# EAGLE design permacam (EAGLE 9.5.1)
AUTHOR: NEAL JACKSON; REV: A; TITLE: PERMAMOTE

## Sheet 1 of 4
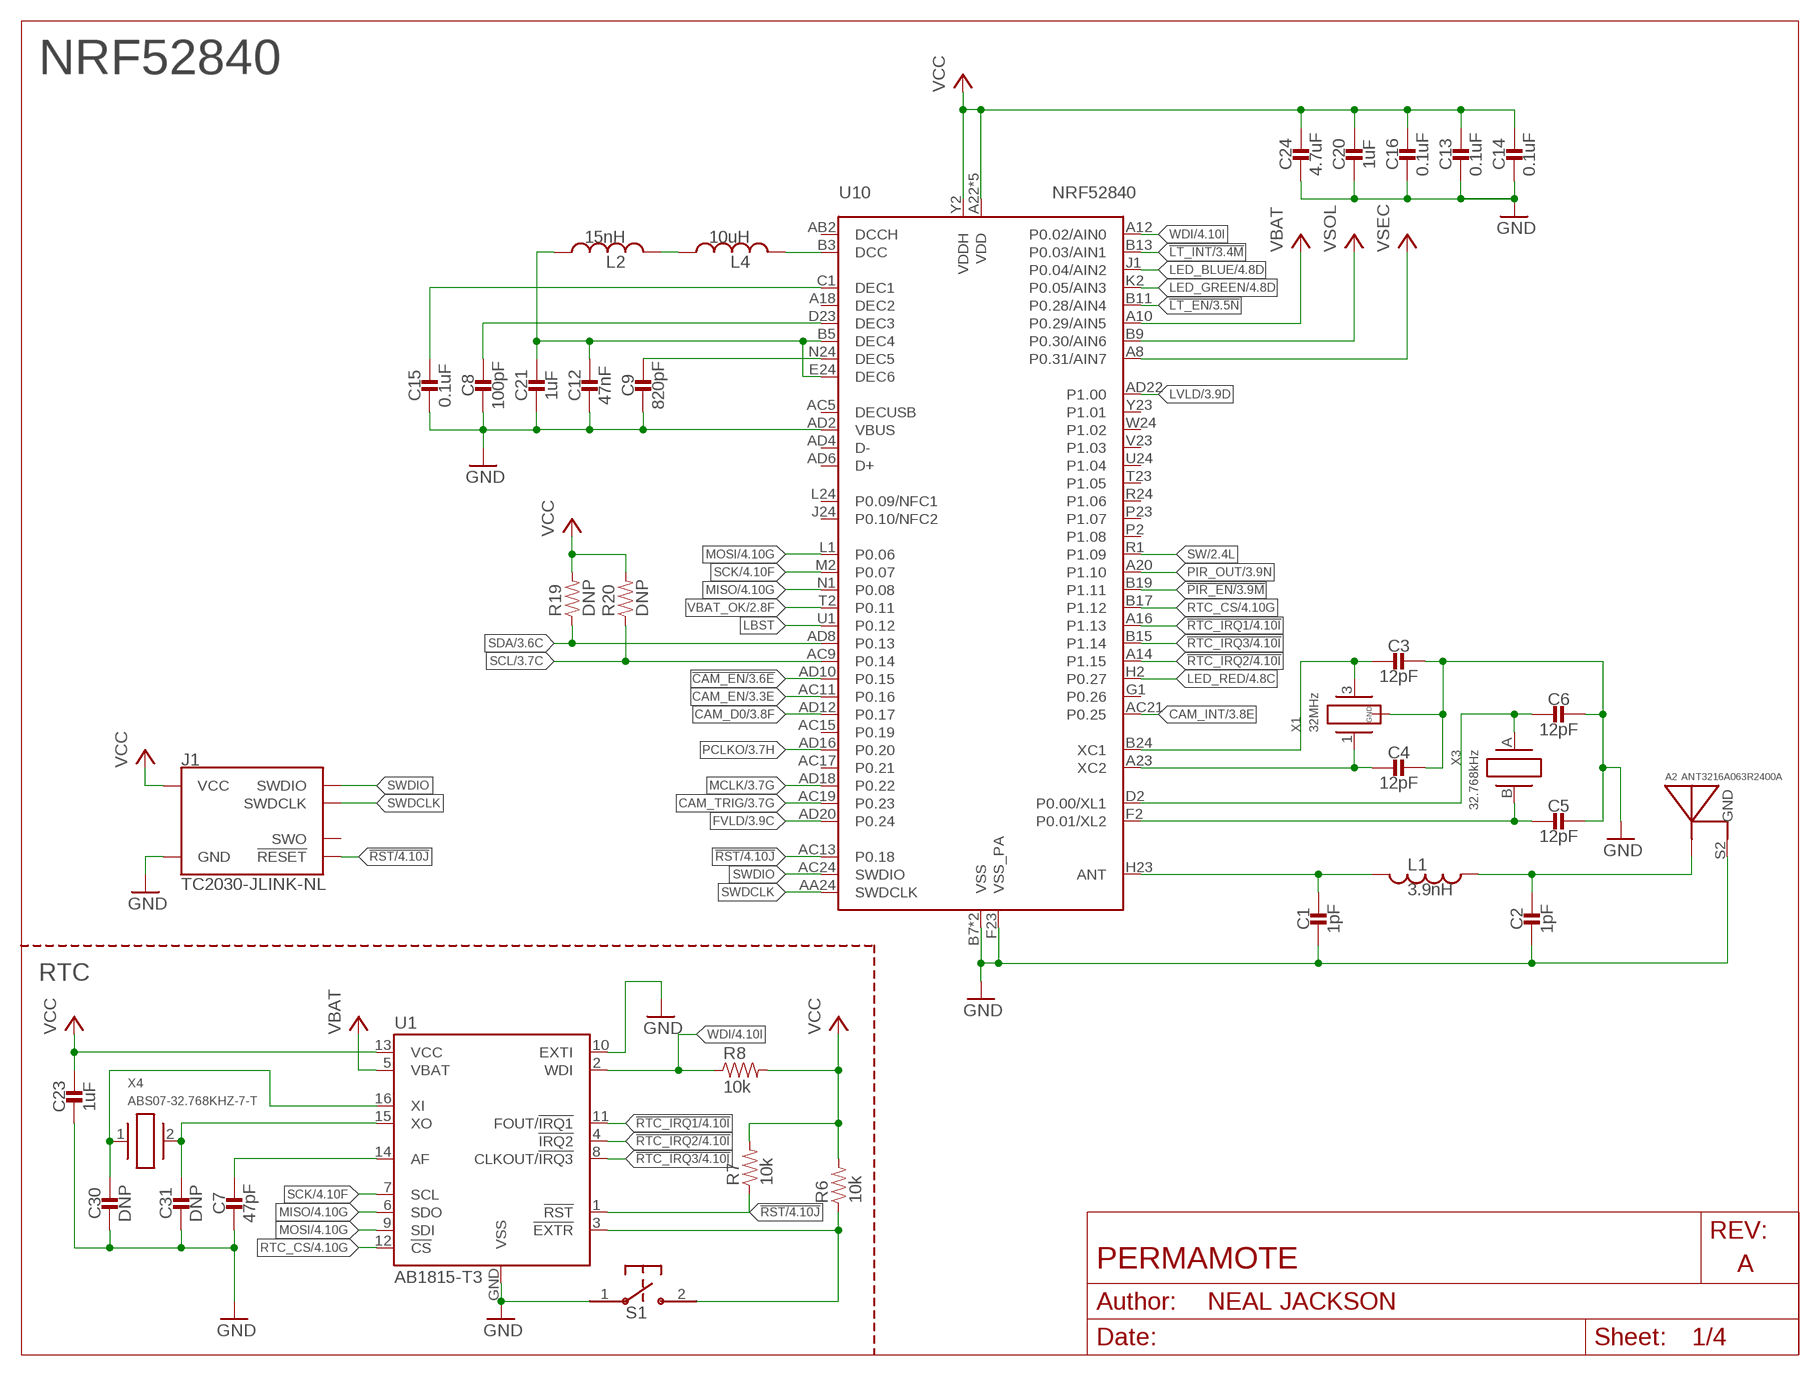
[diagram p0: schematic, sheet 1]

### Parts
A2  ANT3216A063R2400A  [ANT3216A063R2400A]
C1  1pF  CAPACITOR0402_CAP  [0402_CAP]
C2  1pF  CAPACITOR0402_CAP  [0402_CAP]
C3  12pF  CAPACITOR0402_CAP  [0402_CAP]
C4  12pF  CAPACITOR0402_CAP  [0402_CAP]
C5  12pF  CAPACITOR0402_CAP  [0402_CAP]
C6  12pF  CAPACITOR0402_CAP  [0402_CAP]
C7  47pF  CAPACITOR0402_CAP  [0402_CAP]
C8  100pF  CAPACITOR0402_CAP  [0402_CAP]
C9  820pF  CAPACITOR0402_CAP  [0402_CAP]
C12  47nF  CAPACITOR0402_CAP  [0402_CAP]
C13  0.1uF  CAPACITOR0402_CAP  [0402_CAP]
C14  0.1uF  CAPACITOR0402_CAP  [0402_CAP]
C15  0.1uF  CAPACITOR0402_CAP  [0402_CAP]
C16  0.1uF  CAPACITOR0402_CAP  [0402_CAP]
C20  1uF  CAPACITOR0402_CAP  [0402_CAP]
C21  1uF  CAPACITOR0402_CAP  [0402_CAP]
C23  1uF  CAPACITOR0402_CAP  [0402_CAP]
C24  4.7uF  CAPACITOR0402_CAP  [0402_CAP]
C30  DNP  CAPACITOR0402_CAP  [0402_CAP]
C31  DNP  CAPACITOR0402_CAP  [0402_CAP]
J1  TC2030-JLINK-NL  [TC2030-IDC-NL]
L1  3.9nH  INDUCTOR0402  [0402_CAP]
L2  15nH  INDUCTOR0402  [0402_CAP]
L4  10uH  INDUCTOR0603  [0603_CAP]
R6  10k  RESISTOR0402_RES  [0402_RES]
R7  10k  RESISTOR0402_RES  [0402_RES]
R8  10k  RESISTOR0402_RES  [0402_RES]
R19  DNP  RESISTOR0402_RES  [0402_RES]
R20  DNP  RESISTOR0402_RES  [0402_RES]
S1  B3U-1000P  [B3U-1000P]
U1  AB1815-T3  [QFN-16-3MM]
U10  NRF52840  [AQFN73]
X1  32MHz  7V-32.000MAHV-T  [TXC-7V]
X3  32.768kHz  ABS05-32.768KHZ-9-T  [ABS05]
X4  ABS07-32.768KHZ-7-T  [2-SMD]

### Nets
!CAM_EN: U10.AD10(P0.15) ; also sheet 3
!LT_EN: U10.B11(P0.28/AIN4) ; also sheet 3,4
!LT_INT: U10.B13(P0.03/AIN1) ; also sheet 3,4
!PIR_EN: U10.B19(P1.11) ; also sheet 3,4
!RST: J1.3(!RESET) R7.1 U1.1(!RST) U10.AC13(P0.18) ; also sheet 4
!RTC_EXTR: R6.1 S1.2 U1.3(!EXTR)
!RTC_IRQ1: U1.11(FOUT/!IRQ1) U10.A16(P1.13) ; also sheet 4
!RTC_IRQ2: U1.4(!IRQ2) U10.A14(P1.15) ; also sheet 4
!RTC_IRQ3: U1.8(CLKOUT/!IRQ3) U10.B15(P1.14) ; also sheet 4
CAM_D0: U10.AD12(P0.17) ; also sheet 3,4
CAM_EN: U10.AC11(P0.16) ; also sheet 3
CAM_INT: U10.AC21(P0.25) ; also sheet 3
CAM_TRIG: U10.AC19(P0.23) ; also sheet 3
FVLD: U10.AD20(P0.24) ; also sheet 3,4
GND: A2.S2(GND) C1.2 C2.2 C3.1 C4.1 C5.1 C6.1 C7.2 C8.2 C9.2 C12.2 C13.2 C14.2 C15.2 C16.2 C20.2 C21.2 C23.2 C24.2 C30.2 C31.2 J1.5(GND) S1.1 U1.10(EXTI) U1.GND(VSS) U10.AD2(VBUS) U10.B7(VSS) U10.F23(VSS_PA) U10.GND(VSS) X1.2(GND) X1.4(GND) ; also sheet 2,3,4
LBST: U10.U1(P0.12) ; also sheet 2
LED_BLUE: U10.J1(P0.04/AIN2) ; also sheet 4
LED_GREEN: U10.K2(P0.05/AIN3) ; also sheet 4
LED_RED: U10.H2(P0.27) ; also sheet 4
LVLD: U10.AD22(P1.00) ; also sheet 3,4
MCLK: U10.AD18(P0.22) ; also sheet 3,4
MISO: U1.6(SDO) U10.N1(P0.08) ; also sheet 4
MOSI: U1.9(SDI) U10.L1(P0.06) ; also sheet 4
N$1: C9.1 U10.N24(DEC5)
N$2: C15.1 U10.C1(DEC1)
N$3: C12.1 C21.1 L2.1 U10.B5(DEC4) U10.E24(DEC6)
N$4: C8.1 U10.D23(DEC3)
N$5: C1.1 L1.2 U10.H23(ANT)
N$6: A2.S1(ANTENNA) C2.1 L1.1
N$8: C3.2 U10.B24(XC1) X1.3
N$9: C4.2 U10.A23(XC2) X1.1
N$25: C7.1 U1.14(AF)
N$26: C30.1 U1.16(XI) X4.1
N$27: C31.1 U1.15(XO) X4.2
N$44: L4.2 U10.B3(DCC)
N$49: L2.2 L4.1
PCLKO: U10.AD16(P0.20) ; also sheet 3,4
PIR_OUT: U10.A20(P1.10) ; also sheet 3,4
RTC_CS: U1.12(!CS) U10.B17(P1.12) ; also sheet 4
SCK: U1.7(SCL) U10.M2(P0.07) ; also sheet 4
SCL: R20.1 U10.AC9(P0.14) ; also sheet 3,4
SDA: R19.1 U10.AD8(P0.13) ; also sheet 3,4
SW: U10.R1(P1.09) ; also sheet 2,4
SWDCLK: J1.4(SWDCLK) U10.AA24(SWDCLK)
SWDIO: J1.2(SWDIO) U10.AC24(SWDIO)
VBAT: U1.5(VBAT) U10.A10(P0.29/AIN5) ; also sheet 2
VBAT_OK: U10.T2(P0.11) ; also sheet 2
VCC: C13.1 C14.1 C16.1 C20.1 C23.1 C24.1 J1.1(VCC) R6.2 R7.2 R8.2 R19.2 R20.2 U1.13(VCC) U10.A22(VDD) U10.AD14(VDD) U10.AD23(VDD) U10.B1(VDD) U10.W1(VDD) U10.Y2(VDDH) ; also sheet 2,3,4
VSEC: U10.A8(P0.31/AIN7) ; also sheet 2
VSOL: U10.B9(P0.30/AIN6) ; also sheet 2,4
WDI: R8.1 U1.2(WDI) U10.A12(P0.02/AIN0) ; also sheet 4
XL1: C6.2 U10.D2(P0.00/XL1) X3.A
XL2: C5.2 U10.F2(P0.01/XL2) X3.B
Unconnected: J1.6(SWO) U10.A18(DEC2) U10.AB2(DCCH) U10.AC5(DECUSB) U10.AC15(P0.19) U10.AC17(P0.21) U10.AD4(D-) U10.AD6(D+) U10.G1(P0.26) U10.J24(P0.10/NFC2) U10.L24(P0.09/NFC1) U10.P2(P1.08) U10.P23(P1.07) U10.R24(P1.06) U10.T23(P1.05) U10.U24(P1.04) U10.V23(P1.03) U10.W24(P1.02) U10.Y23(P1.01)

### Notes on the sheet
- NRF52840
- RTC

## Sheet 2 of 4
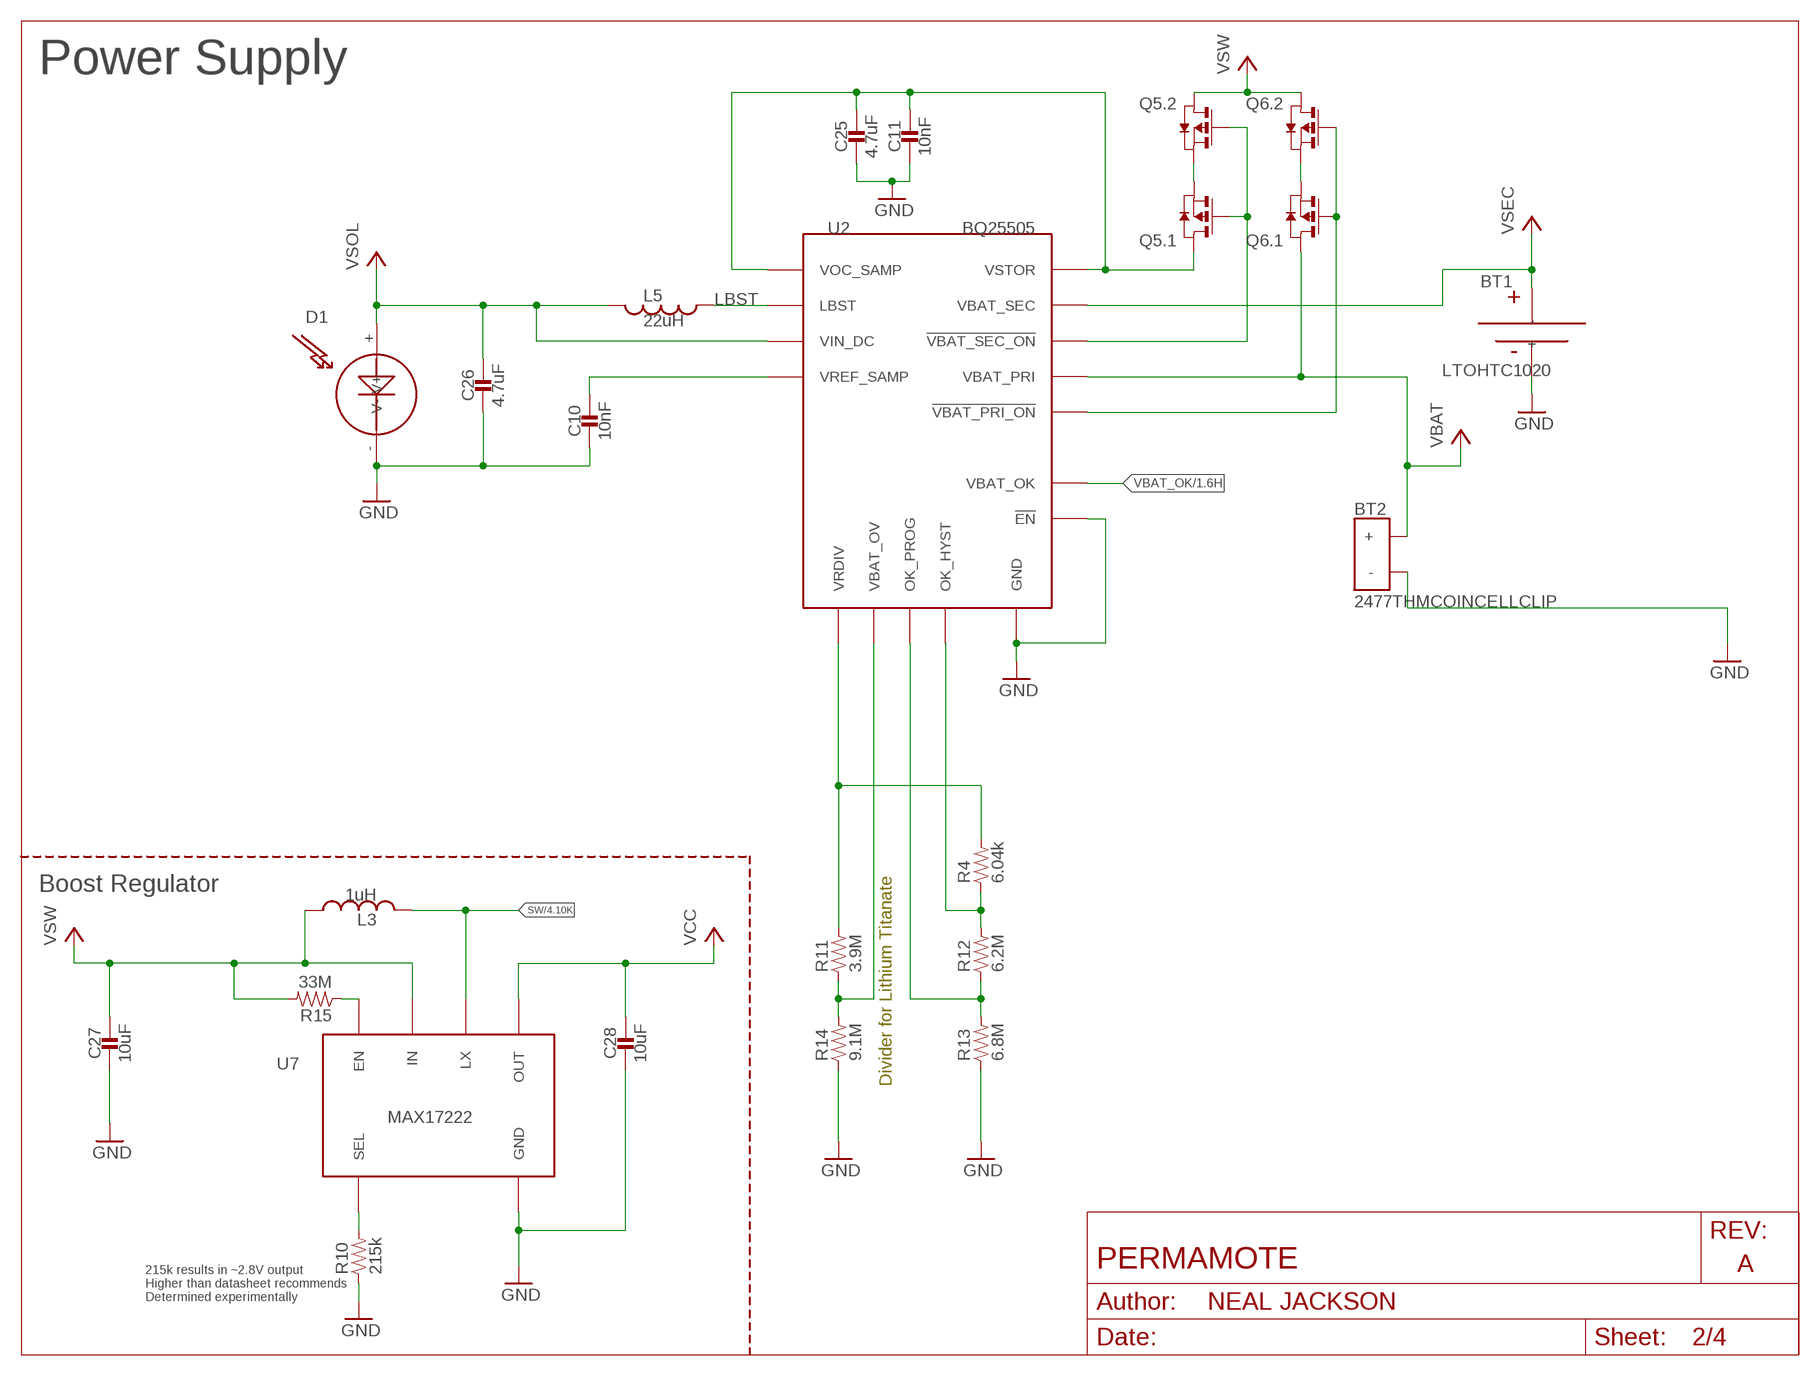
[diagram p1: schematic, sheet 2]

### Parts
BT1  LTOHTC1020  [1020]
BT2  2477THMCOINCELLCLIP  [2477THMCOINCLIP]
C10  10nF  CAPACITOR0402_CAP  [0402_CAP]
C11  10nF  CAPACITOR0402_CAP  [0402_CAP]
C25  4.7uF  CAPACITOR0402_CAP  [0402_CAP]
C26  4.7uF  CAPACITOR0402_CAP  [0402_CAP]
C27  10uF  CAPACITOR0603_CAP  [0603_CAP]
C28  10uF  CAPACITOR0603_CAP  [0603_CAP]
D1  SOLARCELLHOLES  [SOLAR_HOLES]
L3  1uH  INDUCTORIHL  [IHL-1212BZ-11]
L5  22uH  INDUCTOR74437324220  [74437324220]
Q5  PMDXB950UPEL  [XDFN-6]
Q6  PMDXB950UPEL  [XDFN-6]
R4  6.04k  RESISTOR0402_RES  [0402_RES]
R10  215k  RESISTOR0603_RES  [0603-RES]
R11  3.9M  RESISTOR0402_RES  [0402_RES]
R12  6.2M  RESISTOR0402_RES  [0402_RES]
R13  6.8M  RESISTOR0402_RES  [0402_RES]
R14  9.1M  RESISTOR0402_RES  [0402_RES]
R15  33M  RESISTOR0603_RES  [0603-RES]
U2  BQ25505  [S-PVQFN-N20-RGR]
U7  MAX17222  [UDFN-6-MAXIM]

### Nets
!VBAT_PRI_ON: Q6.2(.1:G) Q6.5(.2:G) U2.10(!VBAT_PRI_ON)
!VBAT_SEC_ON: Q5.2(.1:G) Q5.5(.2:G) U2.9(!VBAT_SEC_ON)
GND: BT1.- BT2.GND(-) C10.2 C11.2 C25.2 C26.2 C27.2 C28.2 D1.-(V-) R10.1 R13.1 R14.1 U2.1(GND) U2.5(!EN) U2.6(GND) U2.15(GND) U2.16(GND) U2.17(GND) U2.PAD(GND) U7.3(GND) ; also sheet 1,3,4
LBST: L5.P$1 U2.20(LBST) ; also sheet 1
N$12: R10.2 U7.4(SEL)
N$14: R15.1 U7.6(EN)
N$18: R11.1 R14.2 U2.7(VBAT_OV)
N$32: R4.2 R11.2 U2.8(VRDIV)
N$45: Q5.1(.1:S) Q5.4(.2:S)
N$53: Q6.1(.1:S) Q6.4(.2:S)
N$57: R12.1 R13.2 U2.12(OK_PROG)
N$58: R4.1 R12.2 U2.11(OK_HYST)
SW: L3.P$2 U7.2(LX) ; also sheet 1,4
VBAT: BT2.1(+) BT2.2(+) Q6.6(.1:D) U2.14(VBAT_PRI) ; also sheet 1
VBAT_OK: U2.13(VBAT_OK) ; also sheet 1
VCC: C28.1 U7.1(OUT) ; also sheet 1,3,4
VOC_SAMP_VSTOR: C11.1 C25.1 Q5.6(.1:D) U2.3(VOC_SAMP) U2.19(VSTOR)
VREF_SAMP: C10.1 U2.4(VREF_SAMP)
VSEC: BT1.+ U2.18(VBAT_SEC) ; also sheet 1
VSOL: C26.1 D1.+(V+) L5.P$2 U2.2(VIN_DC) ; also sheet 1,4
VSW: C27.1 L3.P$1 Q5.3(.2:D) Q6.3(.2:D) R15.2 U7.5(IN)

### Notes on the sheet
- Power Supply
- Boost Regulator
- Divider for Lithium Titanate
- 215k results in ~2.8V output
  Higher than datasheet recommends
  Determined experimentally

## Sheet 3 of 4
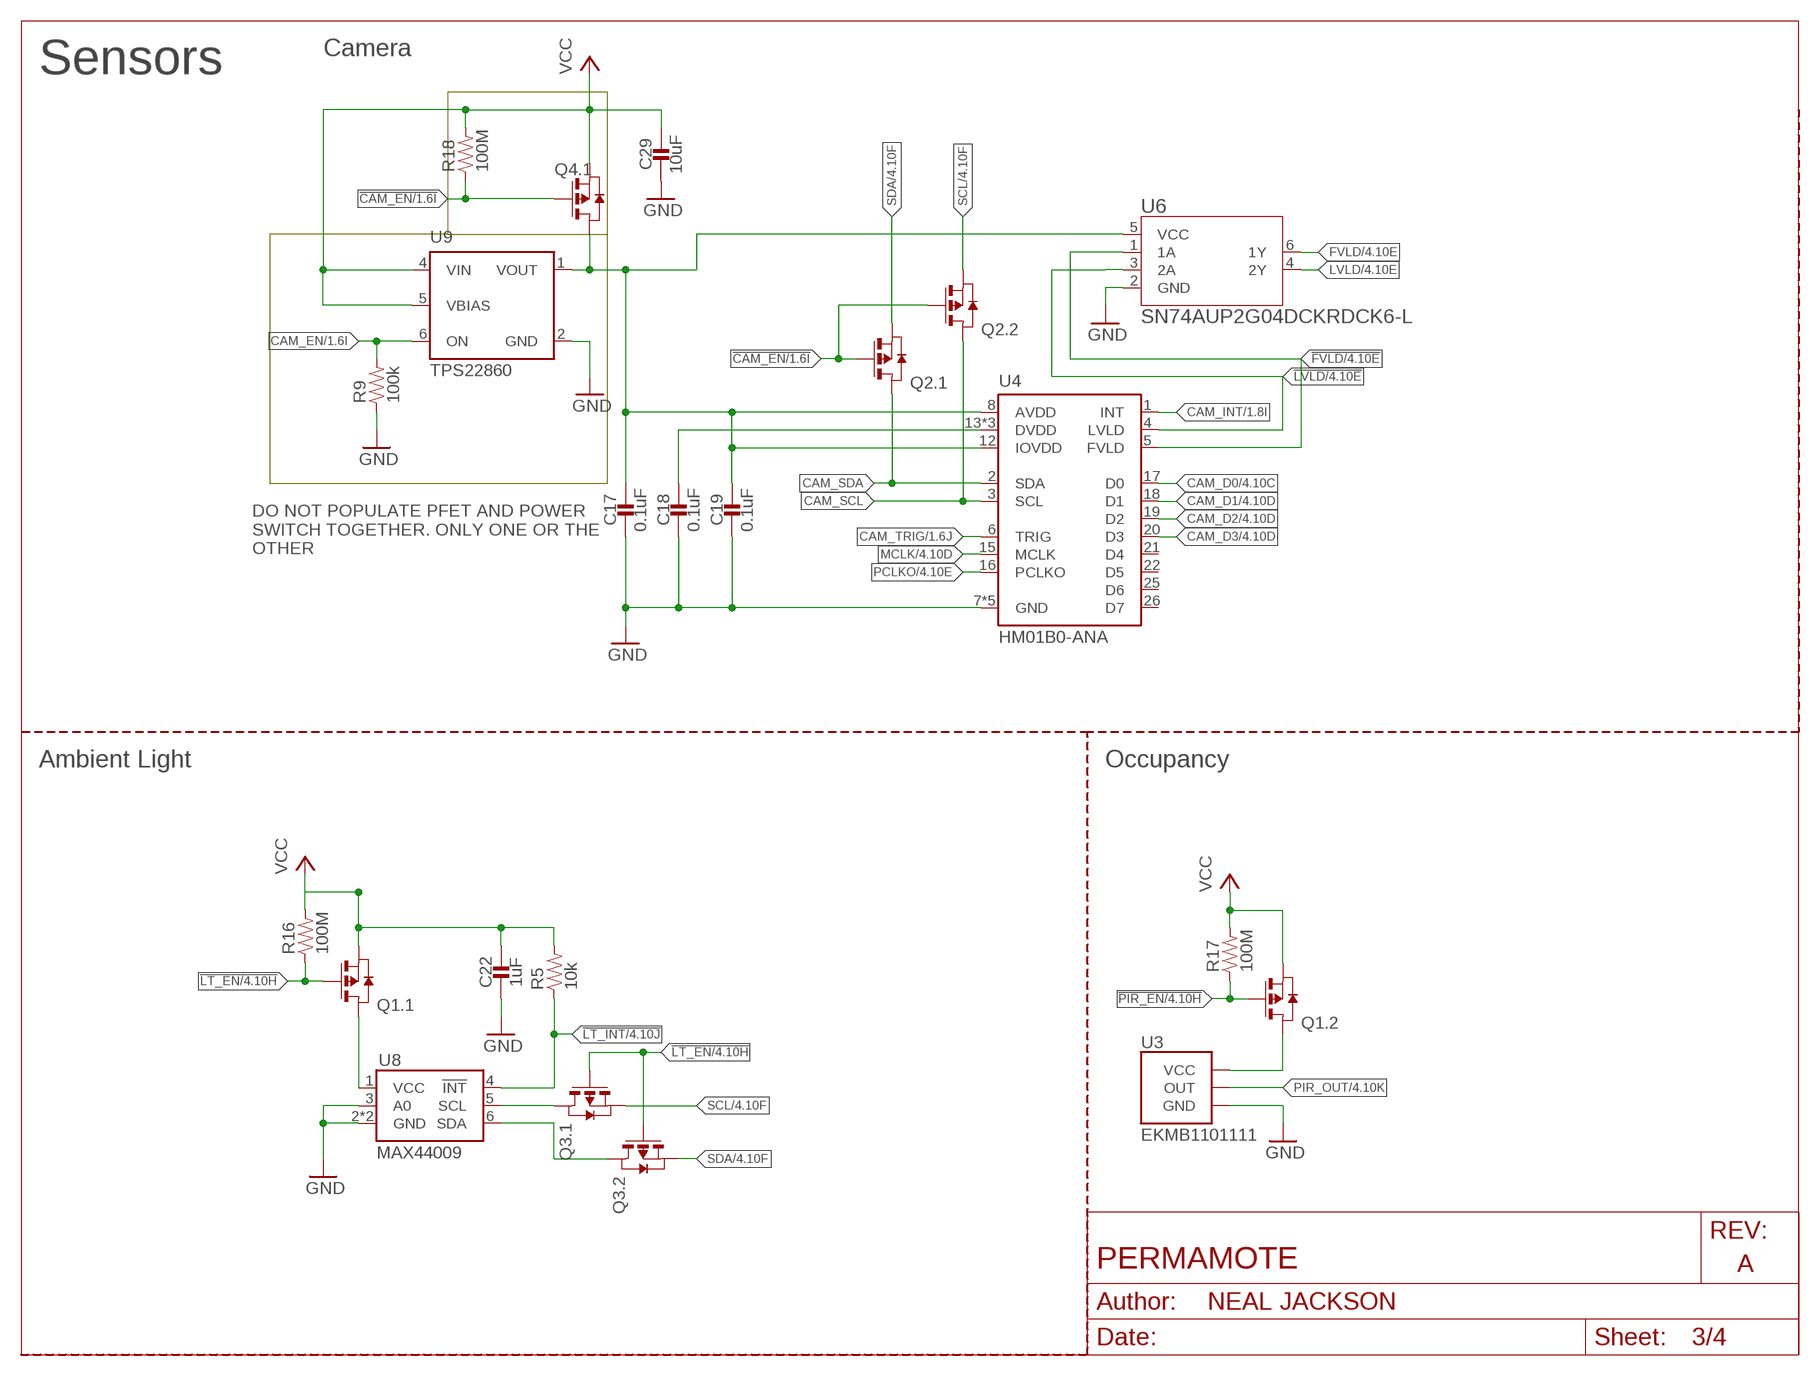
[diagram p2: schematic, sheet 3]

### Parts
C17  0.1uF  CAPACITOR0402_CAP  [0402_CAP]
C18  0.1uF  CAPACITOR0402_CAP  [0402_CAP]
C19  0.1uF  CAPACITOR0402_CAP  [0402_CAP]
C22  1uF  CAPACITOR0402_CAP  [0402_CAP]
C29  10uF  CAPACITOR0603_CAP  [0603_CAP]
Q1  PMDXB950UPEL  [XDFN-6]
Q2  PMDXB950UPEL  [XDFN-6]
Q3  PMDXB950UPEL  [XDFN-6]
Q4  PMDXB950UPEL  [XDFN-6]
R5  10k  RESISTOR0402_RES  [0402_RES]
R9  100k  RESISTOR0402_RES  [0402_RES]
R16  100M  RESISTOR0402_RES  [0402_RES]
R17  100M  RESISTOR0402_RES  [0402_RES]
R18  100M  RESISTOR0402_RES  [0402_RES]
U3  EKMB1101111  [AMN2]
U4  HM01B0-ANA  [NEOPAC-26]
U6  SN74AUP2G04DCKRDCK6-L  [DCK6-L]
U8  MAX44009  [UDFN-6-EXPOSED]
U9  TPS22860  [SOT-23-6]

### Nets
!CAM_EN: Q2.2(.1:G) Q2.5(.2:G) Q4.2(.1:G) R18.1 ; also sheet 1
!FVLD: U4.5(FVLD) U6.1(1A) ; also sheet 4
!LT_EN: Q1.2(.1:G) Q3.2(.1:G) Q3.5(.2:G) R16.1 ; also sheet 1,4
!LT_INT: R5.1 U8.4(!INT) ; also sheet 1,4
!LVLD: U4.4(LVLD) U6.3(2A) ; also sheet 4
!PIR_EN: Q1.5(.2:G) R17.1 ; also sheet 1,4
CAM_D0: U4.17(D0) ; also sheet 1,4
CAM_D1: U4.18(D1) ; also sheet 4
CAM_D2: U4.19(D2) ; also sheet 4
CAM_D3: U4.20(D3) ; also sheet 4
CAM_EN: R9.2 U9.6(ON) ; also sheet 1
CAM_INT: U4.1(INT) ; also sheet 1
CAM_SCL: Q2.3(.2:D) U4.3(SCL)
CAM_SDA: Q2.6(.1:D) U4.2(SDA)
CAM_TRIG: U4.6(TRIG) ; also sheet 1
FVLD: U6.6(1Y) ; also sheet 1,4
GND: C17.2 C18.2 C19.2 C22.2 C29.2 R9.1 U3.GND U4.7(GND) U4.9(GND) U4.10(GND) U4.11(GND) U4.24(GND) U6.2(GND) U8.2(GND) U8.3(A0) U8.EP(GND) U9.2(GND) ; also sheet 1,2,4
LVLD: U6.4(2Y) ; also sheet 1,4
MCLK: U4.15(MCLK) ; also sheet 1,4
N$10: C18.1 U4.13(DVDD) U4.14(DVDD) U4.23(DVDD)
N$13: C17.1 C19.1 Q4.6(.1:D) U4.8(AVDD) U4.12(IOVDD) U6.5(VCC) U9.1(VOUT)
N$20: Q1.6(.1:D) U8.1(VCC)
N$23: Q1.3(.2:D) U3.VCC
N$51: Q3.3(.2:D) U8.6(SDA)
N$52: Q3.6(.1:D) U8.5(SCL)
PCLKO: U4.16(PCLKO) ; also sheet 1,4
PIR_OUT: U3.OUT ; also sheet 1,4
SCL: Q2.4(.2:S) Q3.1(.1:S) ; also sheet 1,4
SDA: Q2.1(.1:S) Q3.4(.2:S) ; also sheet 1,4
VCC: C22.1 C29.1 Q1.1(.1:S) Q1.4(.2:S) Q4.1(.1:S) R5.2 R16.2 R17.2 R18.2 U9.4(VIN) U9.5(VBIAS) ; also sheet 1,2,4
Unconnected: Q4.3(.2:D) Q4.4(.2:S) Q4.5(.2:G) U4.21(D4) U4.22(D5) U4.25(D6) U4.26(D7)

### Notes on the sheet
- Camera
- Sensors
- DO NOT POPULATE PFET AND POWER
  SWITCH TOGETHER. ONLY ONE OR THE
  OTHER
- Ambient Light | Occupancy

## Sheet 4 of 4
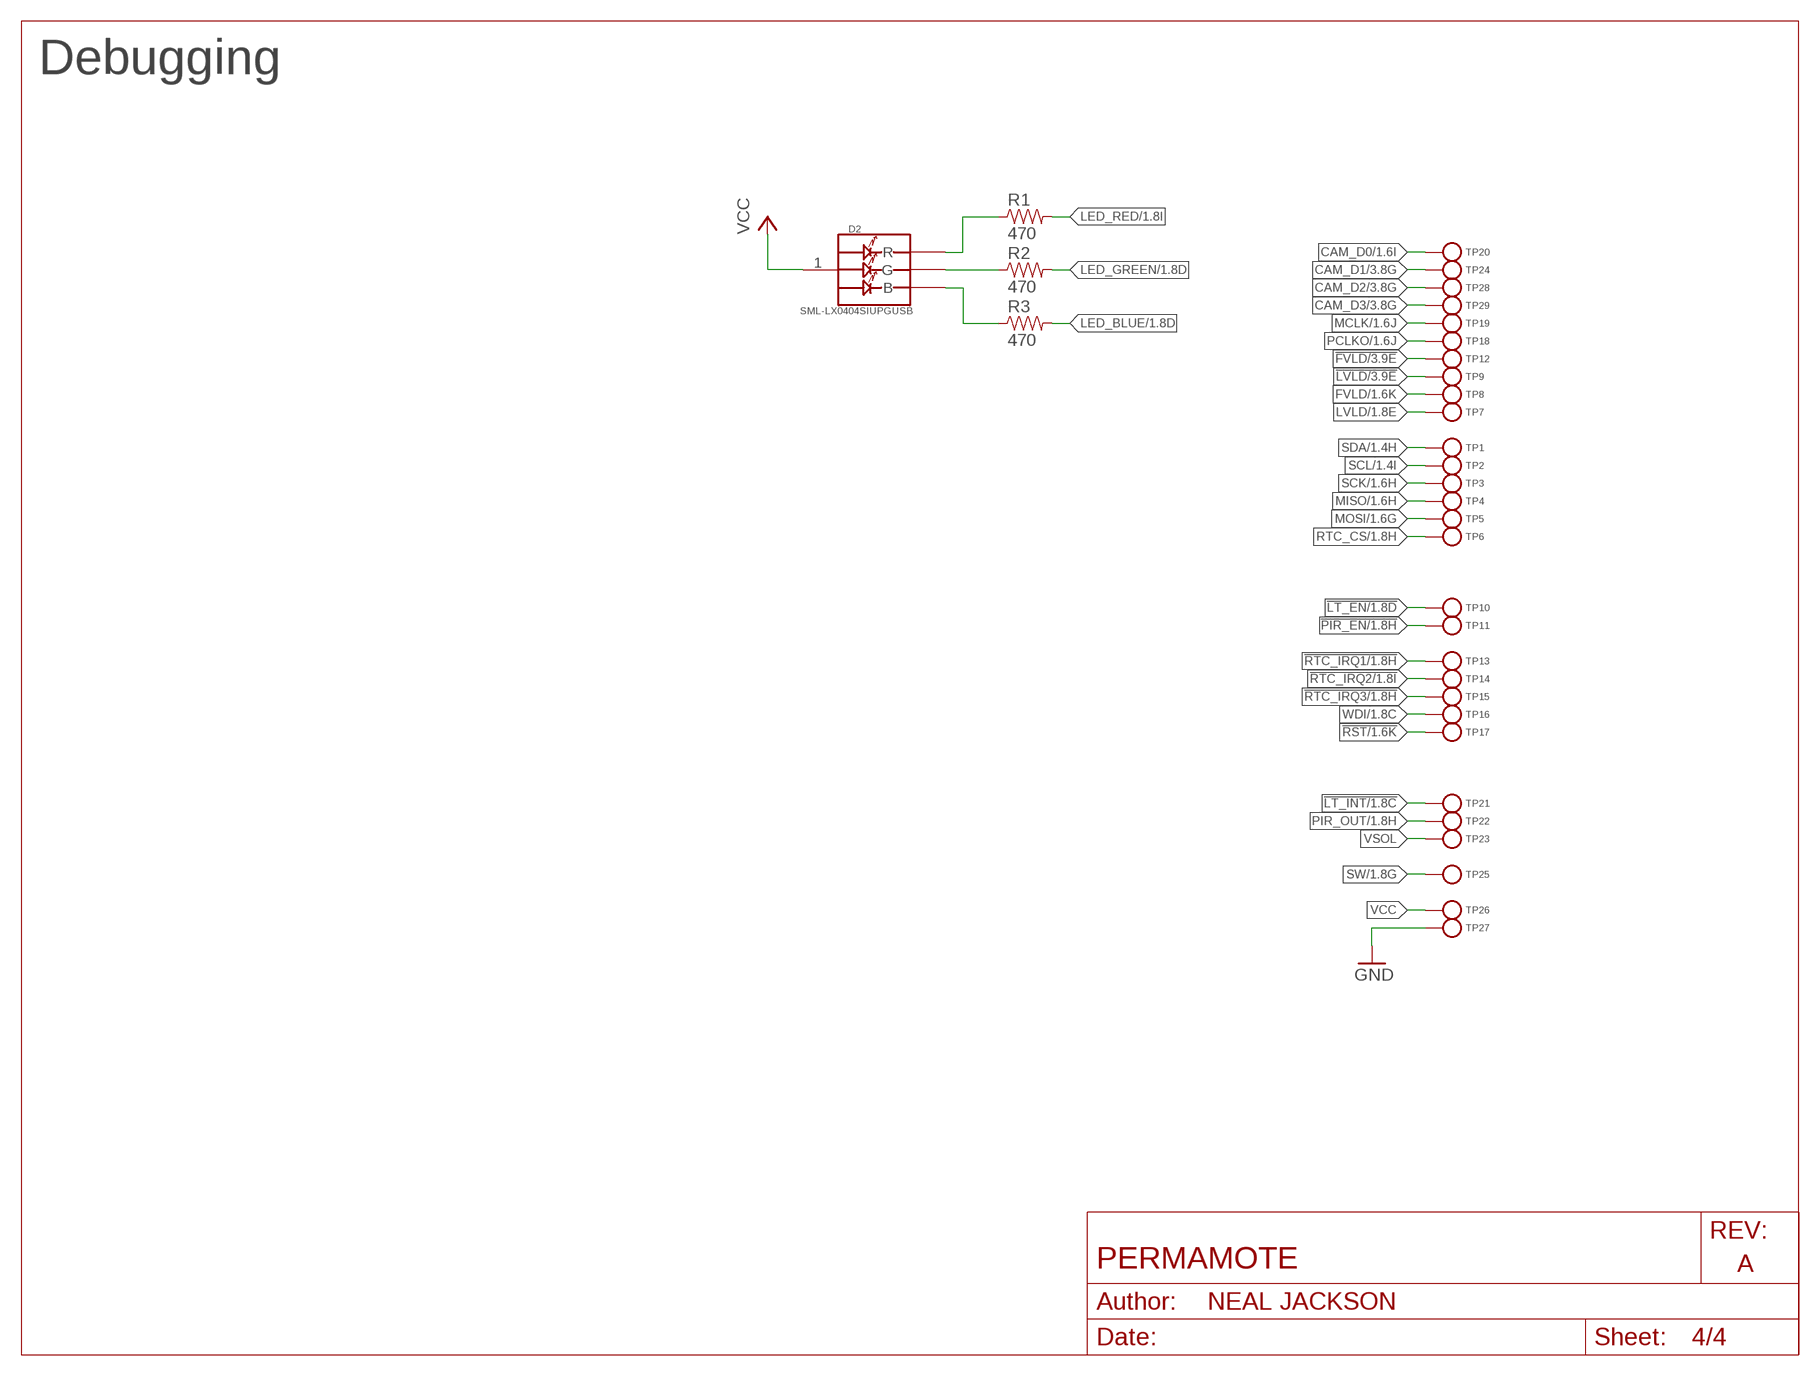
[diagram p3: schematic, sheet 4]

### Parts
D2  SML-LX0404SIUPGUSB  [1MM_SQ_4PAD]
R1  470  RESISTOR0402_RES  [0402_RES]
R2  470  RESISTOR0402_RES  [0402_RES]
R3  470  RESISTOR0402_RES  [0402_RES]
TP1  TEST-POINT  [PAD.03X.03]
TP2  TEST-POINT  [PAD.03X.03]
TP3  TEST-POINT  [PAD.03X.03]
TP4  TEST-POINT  [PAD.03X.03]
TP5  TEST-POINT  [PAD.03X.03]
TP6  TEST-POINT  [PAD.03X.03]
TP7  TEST-POINT  [PAD.03X.03]
TP8  TEST-POINT  [PAD.03X.03]
TP9  TEST-POINT  [PAD.03X.03]
TP10  TEST-POINT  [PAD.03X.03]
TP11  TEST-POINT  [PAD.03X.03]
TP12  TEST-POINT  [PAD.03X.03]
TP13  TEST-POINT  [PAD.03X.03]
TP14  TEST-POINT  [PAD.03X.03]
TP15  TEST-POINT  [PAD.03X.03]
TP16  TEST-POINT  [PAD.03X.03]
TP17  TEST-POINT  [PAD.03X.03]
TP18  TEST-POINT  [PAD.03X.03]
TP19  TEST-POINT  [PAD.03X.03]
TP20  TEST-POINT  [PAD.03X.03]
TP21  TEST-POINT  [PAD.03X.03]
TP22  TEST-POINT  [PAD.03X.03]
TP23  TEST-POINT  [PAD.03X.03]
TP24  TEST-POINT  [PAD.03X.03]
TP25  TEST-POINT  [PAD.03X.03]
TP26  TEST-POINT  [PAD.03X.03]
TP27  TEST-POINT  [PAD.03X.03]
TP28  TEST-POINT  [PAD.03X.03]
TP29  TEST-POINT  [PAD.03X.03]

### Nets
!FVLD: TP12.P$1(TESTPOINT) ; also sheet 3
!LT_EN: TP10.P$1(TESTPOINT) ; also sheet 1,3
!LT_INT: TP21.P$1(TESTPOINT) ; also sheet 1,3
!LVLD: TP9.P$1(TESTPOINT) ; also sheet 3
!PIR_EN: TP11.P$1(TESTPOINT) ; also sheet 1,3
!RST: TP17.P$1(TESTPOINT) ; also sheet 1
!RTC_IRQ1: TP13.P$1(TESTPOINT) ; also sheet 1
!RTC_IRQ2: TP14.P$1(TESTPOINT) ; also sheet 1
!RTC_IRQ3: TP15.P$1(TESTPOINT) ; also sheet 1
CAM_D0: TP20.P$1(TESTPOINT) ; also sheet 1,3
CAM_D1: TP24.P$1(TESTPOINT) ; also sheet 3
CAM_D2: TP28.P$1(TESTPOINT) ; also sheet 3
CAM_D3: TP29.P$1(TESTPOINT) ; also sheet 3
FVLD: TP8.P$1(TESTPOINT) ; also sheet 1,3
GND: TP27.P$1(TESTPOINT) ; also sheet 1,2,3
LED_BLUE: R3.2 ; also sheet 1
LED_GREEN: R2.2 ; also sheet 1
LED_RED: R1.2 ; also sheet 1
LVLD: TP7.P$1(TESTPOINT) ; also sheet 1,3
MCLK: TP19.P$1(TESTPOINT) ; also sheet 1,3
MISO: TP4.P$1(TESTPOINT) ; also sheet 1
MOSI: TP5.P$1(TESTPOINT) ; also sheet 1
N$15: D2.2(R) R1.1
N$17: D2.4(G) R2.1
N$19: D2.3(B) R3.1
PCLKO: TP18.P$1(TESTPOINT) ; also sheet 1,3
PIR_OUT: TP22.P$1(TESTPOINT) ; also sheet 1,3
RTC_CS: TP6.P$1(TESTPOINT) ; also sheet 1
SCK: TP3.P$1(TESTPOINT) ; also sheet 1
SCL: TP2.P$1(TESTPOINT) ; also sheet 1,3
SDA: TP1.P$1(TESTPOINT) ; also sheet 1,3
SW: TP25.P$1(TESTPOINT) ; also sheet 1,2
VCC: D2.1(VDD) TP26.P$1(TESTPOINT) ; also sheet 1,2,3
VSOL: TP23.P$1(TESTPOINT) ; also sheet 1,2
WDI: TP16.P$1(TESTPOINT) ; also sheet 1

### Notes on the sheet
- Debugging

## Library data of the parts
A2 = chips:ANT3216A063R2400A: Yageo 2.4GHz; DIGIKEY: 311-1542-1-ND; MANUFACTURER: YAGEO; MPN: ANT3216A063R2400A
BT1 = batteries:LTOHTC
BT2 = batteries:2477THMCOINCELLCLIP: Battery clip for 2477 Coin Cell; DIGIKEY: BAT-HLD-001-THM-ND; MANUFACTURER: Keystone; MPN: BAT-HLD-001-THM
C1 C2 = passives:CAPACITOR: SMD Capacitor; DIGIKEY: 1276-1595-1-ND; MPN: CL05C010CB5NNNC
C3-C6 = passives:CAPACITOR: SMD Capacitor; DIGIKEY: 490-6197-1-ND; MPN: GRM1555C1H120GA01D
C7 = passives:CAPACITOR: SMD Capacitor; DIGIKEY: 490-5942-1-ND; MPN: GRM1555C1H470JA01D
C8 = passives:CAPACITOR: SMD Capacitor; DIGIKEY: 490-5922-1-ND; MPN: GRM1555C1H101JA01D
C9 = passives:CAPACITOR: SMD Capacitor; DIGIKEY: 1276-6535-1-ND; MPN: CL05B821KO5NNNC
C10 C11 = passives:CAPACITOR: SMD Capacitor; DIGIKEY: 490-4516-1-ND; MPN: GRM155R71H103KA88D
C12 = passives:CAPACITOR: SMD Capacitor; DIGIKEY: 445-1264-1-ND; MPN: C1005X7R1C473K050BC
C13-C19 = passives:CAPACITOR: SMD Capacitor; DIGIKEY: 490-6328-1-ND; MPN: GRM155R71C104KA88J
C20-C23 = passives:CAPACITOR: SMD Capacitor; DIGIKEY: 490-7195-1-ND; MPN: GRM155R70G105KA12D
C24-C26 = passives:CAPACITOR: SMD Capacitor; DIGIKEY: 445-5947-1-ND; MPN: C1005X5R0J475K050BC
C27-C29 = passives:CAPACITOR: SMD Capacitor; DIGIKEY: 490-3896-1-ND; MPN: GRM188R60J106ME47D
C30 C31 = passives:CAPACITOR: SMD Capacitor
D1 = permamote:SOLARCELL: Generic solar cell; DIGIKEY: 869-1001-ND; MPN: AM-1454CA
D2 = leds:SML-LX0404SIUPGUSB: 1mm^2 RGB LED; DIGIKEY: 67-2125-1-ND; MANUFACTURER: Lumex Opto; MPN: SML-LX0404SIUPGUSB
J1 = connector:TC2030-JLINK
L1 = passives:INDUCTOR: A very specific inductor; DIGIKEY: 490-1131-1-ND; MPN: LQP15MN3N9B02D
L2 = passives:INDUCTOR: A very specific inductor; DIGIKEY: 587-1521-1-ND; MPN: HK100515NJ-T
L3 = passives:INDUCTOR: A very specific inductor; DIGIKEY: 541-1319-1-ND; MANUFACTURER: Vishay Dale; MPN: IHLP1212BZER1R0M11
L4 = passives:INDUCTOR: A very specific inductor; DIGIKEY: 490-4025-1-ND; MPN: LQM18FN100M00D
L5 = passives:INDUCTOR: A very specific inductor; DIGIKEY: 732-3340-1-ND; MPN: 74437324220
Q1-Q6 = fets:PMDXB950UPEL: 20 V 500mA, dual P-channel Trench MOSFET; DIGIKEY: 1727-2601-1-ND; MANUFACTURER: NEXPERIA; MPN: PMDXB950UPELZ
R1-R3 = passives:RESISTOR: Resistor; DIGIKEY: 311-470JRCT-ND; MPN: RC0402JR-07470RL
R4 = passives:RESISTOR: Resistor; DIGIKEY: YAG2293CT-ND; MPN: RC0402FR-076K04L
R5-R8 = passives:RESISTOR: Resistor; DIGIKEY: 311-10KJRCT-ND; MPN: RC0402JR-0710KL
R9 = passives:RESISTOR: Resistor; DIGIKEY: 311-100KJRCT-ND; MPN: RC0402JR-07100KL
R10 = passives:RESISTOR: Resistor; DIGIKEY: YAG3055CT-ND; MPN: RC0402FR-07215KL
R11 = passives:RESISTOR: Resistor; DIGIKEY: YAG3301CT-ND; MPN: RC0402JR-073M9L
R12 = passives:RESISTOR: Resistor; DIGIKEY: YAG3309CT-ND; MPN: RC0402JR-076M2L
R13 = passives:RESISTOR: Resistor; DIGIKEY: YAG3310CT-ND; MPN: RC0402JR-076M8L
R14 = passives:RESISTOR: Resistor; DIGIKEY: YAG3322CT-ND; MPN: RC0402JR-079M1L
R15 = passives:RESISTOR: Resistor; DIGIKEY: HMC0603JT33M0CT-ND; MPN: HMC0603JT33M0
R16-R18 = passives:RESISTOR: Resistor; DIGIKEY: 541-100MAHCT-ND; MPN: HMC0402JT100M
R19 R20 = passives:RESISTOR: Resistor
S1 = switches:B3U: Switch; DIGIKEY: SW1020CT-ND; MANUFACTURER: Omron; MPN: B3U-1000P
TP1-TP29 = headers:TEST-POINT
U1 = chips:AB1815-T3: Ultra-low current RTC. 55nA quiescent @ 3V. 1.5-3.6V input.; DIGIKEY: 535-11936-1-ND; MANUFACTURER: Abracon; MPN: AB1815-T3
U2 = chips:BQ25505: EH front end for switching between primary and secondary cells; DIGIKEY: 296-37078-1-ND; MANUFACTURER: TI; MPN: BQ25505RGRR
U3 = chips:EKMB: Passive infrared human detection sensor with built-in amp.; DIGIKEY: 255-3065-ND; MANUFACTURER: PANASONIC; MPN: EKMB1101111
U4 = chips:HM01B0: ultra low power CMOS Image Sensor 320 x 320
U6 = chips:SN74AUP2G04DCKR; MANUFACTURER_PART_NUMBER: SN74AUP2G04DCKR; VENDOR: Texas Instruments
U7 = chips:MAX17222: Very high efficiency, very low power boost converter suitable for EH applications; DIGIKEY: MAX17222ELT+TCT-ND; MANUFACTURER: MAXIM INTEGRATED; MPN: MAX17222ELT+T
U8 = chips:MAX44009: low power ambient light sensor; DIGIKEY: MAX44009EDT+TCT-ND; MANUFACTURER: MAXIM; MPN: MAX44009EDT+T
U9 = chips:TPS22860: Ultra-Low Leakage Load Switch; DIGIKEY: 296-43982-1-ND; MPN: TPS22860DBVR
U10 = chips:NRF52840: ultra-low power 2.4 GHz wireless system on chip (SoC) integrating a multiprotocol 2.4 GHz transceiver, an ARM® Cortex®-M4F CPU.; DIGIKEY: 1490-1071-1-ND; MANUFACTURER: NORIDIC SEMICONDUCTOR; MPN: NRF52840
X1 = crystals:7V: TXC CRYSTAL SMD; DIGIKEY: 887-2568-1-ND; MANUFACTURER: TXC CORPORATION; MPN: 7M-32.000MAHV-T
X3 = crystals:ABS05-32.768KHZ: 32.768kHz Crystal; DIGIKEY: 535-11897-1-ND; MANUFACTURER: Abracon; MPN: ABS05-32.768KHZ-9-T
X4 = crystals:ABS07-32.768KHZ: 32.768kHz Crystal; DIGIKEY: 535-9543-1-ND; MANUFACTURER: ABRACON; MPN: ABS07-32.768KHZ-7-T

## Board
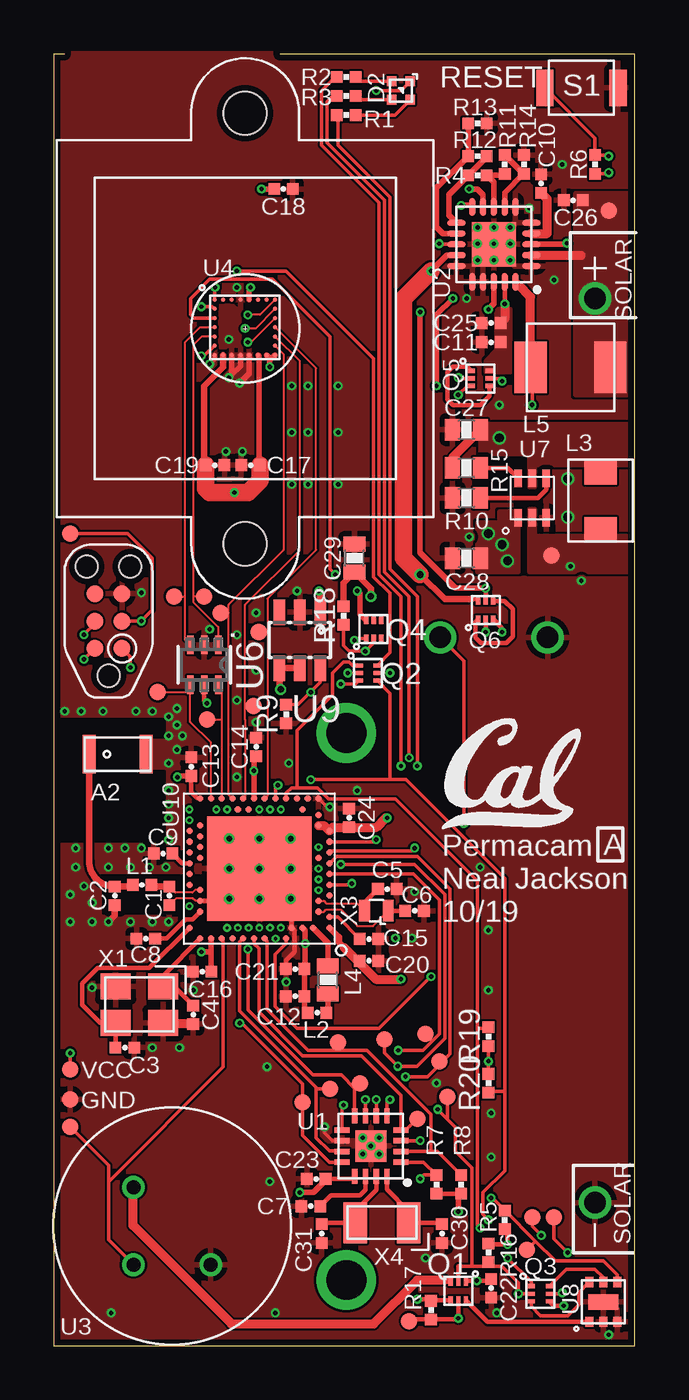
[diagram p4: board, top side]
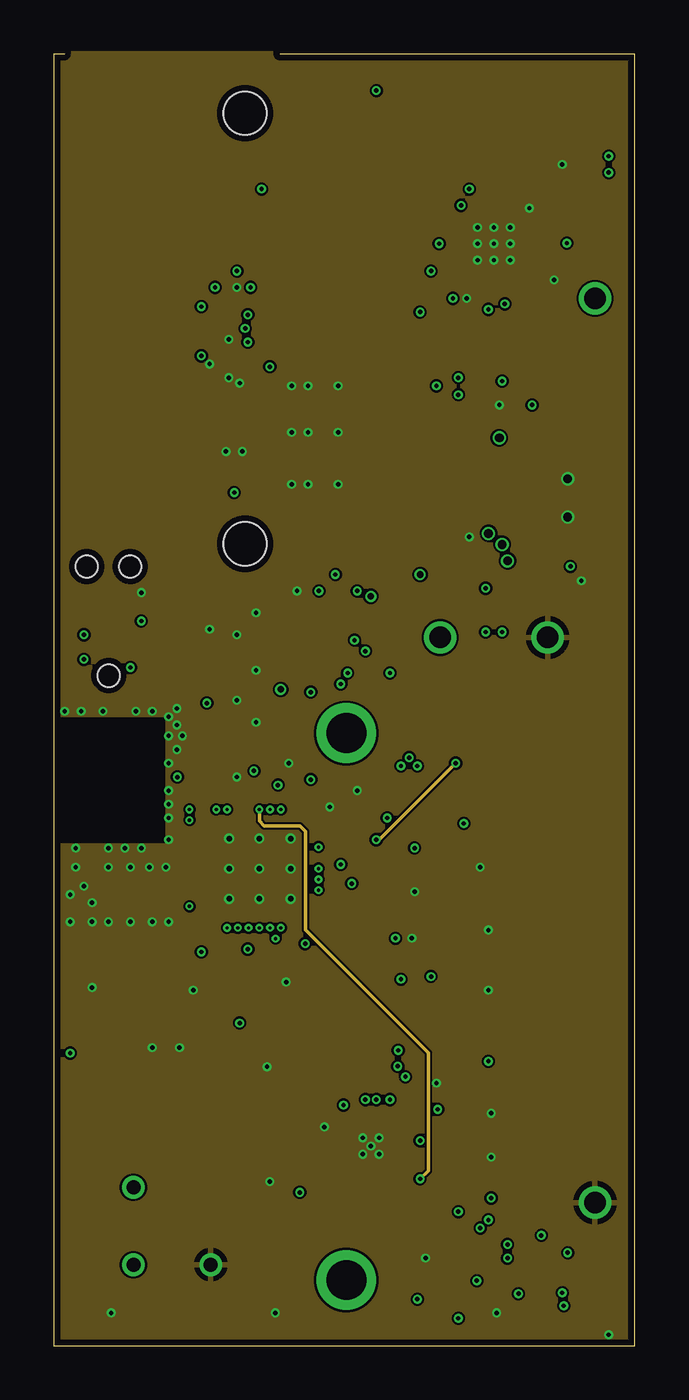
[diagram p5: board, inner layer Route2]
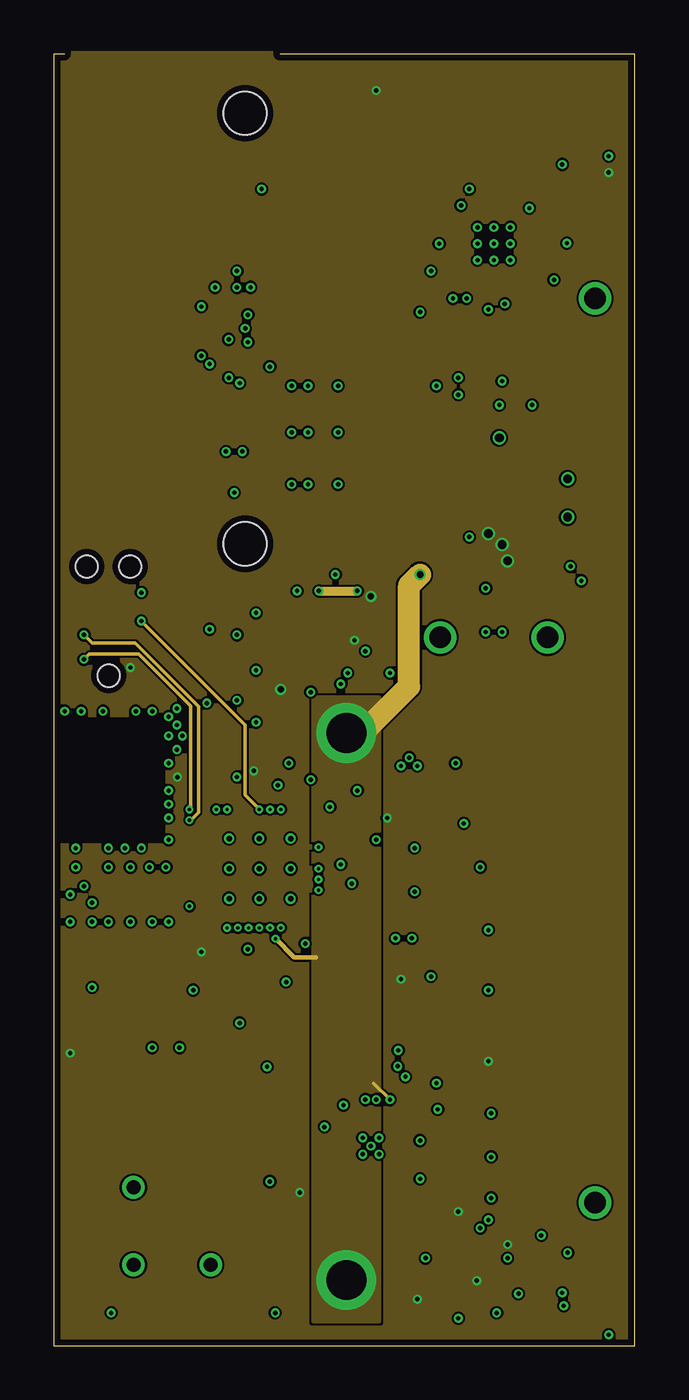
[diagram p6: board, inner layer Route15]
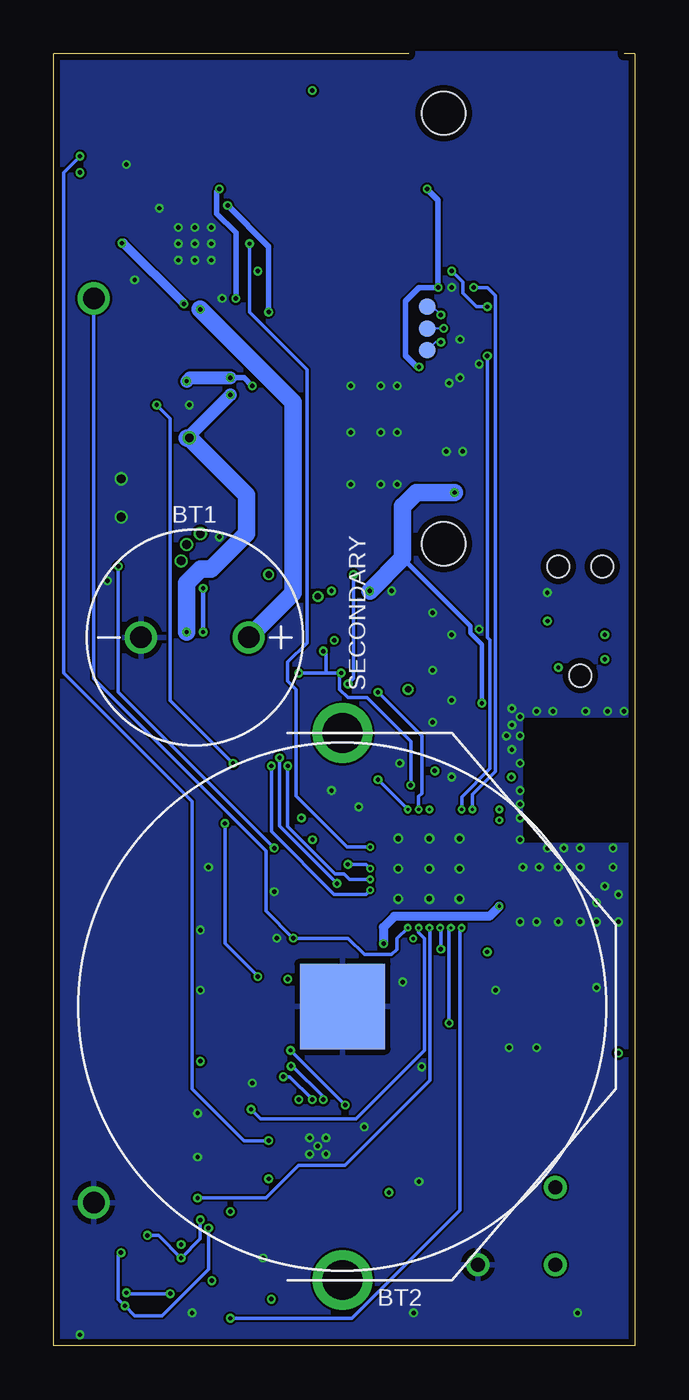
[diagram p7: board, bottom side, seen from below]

Size 27 x 60 mm. Coordinates in mm from the lower left corner, seen from the top.
Outline: 0.5,60 0,60 0,0 27,0 27,60 10.5,60
Copper layers (1+2*15+16): Top 0.0178mm / dielectric 59mil / Route2 0.0356mm / dielectric 0.1499mm / Route15 0.0356mm / dielectric 0.2007mm / Bottom 0.0178mm
Design rules "quickturn_co_kr_1oz_4lyr *": minimum track width 4mil, minimum drill 8mil, track to track 4mil, track to pad 4mil, pad to pad 4mil, via to via 4mil, smd to smd 4mil, copper to edge 12mil, drill to drill 12mil, minimum pad ring 8mil, minimum via ring 4mil, stop-mask expansion 3mil, vias tented up to drill 50mil, thermal gap 10mil
tRestrict: area 25.8,0.9 to 25.9,1.4

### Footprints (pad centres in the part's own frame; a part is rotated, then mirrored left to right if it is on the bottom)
ANT3216A063R2400A = smd 0.6 x 1.8: S1 -1.325,0; S2 1.325,0
1020 = drill 1: + -2.5,0; - 2.5,0
2477THMCOINCLIP = drill 1.854: 1 -12.7,0; 2 12.7,0 | smd 3.962 x 3.962: GND 0,0
0402_CAP = smd 0.536 x 0.546: 1 -0.433,0; 2 0.433,0
0603_CAP = smd 0.7 x 1: 1 -0.65,0; 2 0.65,0
SOLAR_HOLES = drill 1: + 0,0; - 42,0
1MM_SQ_4PAD = smd 0.457 x 0.457: 1 0.432,0.432; 2 0.432,-0.432; 3 -0.432,-0.432; 4 -0.432,0.432
TC2030-IDC-NL = smd 0.787 x 0.787: 1 -1.27,-0.635; 2 -1.27,0.635; 3 0,-0.635; 4 0,0.635; 5 1.27,-0.635; 6 1.27,0.635 | hole 1.016: -2.54,0; 2.54,1.016; 2.54,-1.016
IHL-1212BZ-11 = smd 1.2 x 1.5: P$1 -1.35,0; P$2 1.35,0
74437324220 = smd 1.5 x 2.4: P$1 1.85,0; P$2 -1.85,0
XDFN-6 = smd 0.35 x 0.2: 1 -0.425,0.35; 2 -0.425,0; 3 -0.425,-0.35; 4 0.425,-0.35; 5 0.425,0; 6 0.425,0.35
0402_RES = smd 0.536 x 0.546: 1 -0.433,0; 2 0.433,0
0603-RES = smd 0.7 x 1: 1 -0.65,0; 2 0.65,0
B3U-1000P = smd 0.8 x 1.7: 1 -1.7,0; 2 1.7,0
PAD.03X.03 = smd 0.762 x 0.762: P$1 0,0
QFN-16-3MM = smd 0.7 x 0.25: 1 -1.4,0.75; 2 -1.4,0.25; 3 -1.4,-0.25; 4 -1.4,-0.75; 9 1.35,-0.75; 10 1.35,-0.25; 11 1.35,0.25; 12 1.35,0.75 | smd 0.25 x 0.7: 5 -0.75,-1.4; 6 -0.25,-1.4; 7 0.25,-1.4; 8 0.75,-1.4; 13 0.75,1.4; 14 0.25,1.4; 15 -0.25,1.4; 16 -0.75,1.4 | smd 1.45 x 1.45: GND 0,0
S-PVQFN-N20-RGR = smd 0.28 x 0.85: 1 -1,-1.74; 2 -0.5,-1.74; 3 0,-1.74; 4 0.5,-1.74; 5 1,-1.74; 11 1,1.74; 12 0.5,1.74; 13 0,1.74; 14 -0.5,1.74; 15 -1,1.74 | smd 0.85 x 0.28: 6 1.74,-1; 7 1.74,-0.5; 8 1.74,0; 9 1.74,0.5; 10 1.74,1; 16 -1.74,1; 17 -1.74,0.5; 18 -1.74,0; 19 -1.74,-0.5; 20 -1.74,-1 | smd 2.05 x 2.05: PAD 0,0
AMN2 = drill 0.65: GND 1.796,-1.796; OUT -1.796,-1.796; VCC -1.796,1.796
NEOPAC-26 = smd 0.22 x 0.22: 1 -1.427,1.346; 2 -1.427,0.916; 3 -1.427,0.487; 4 -1.427,0.058; 5 -1.427,-0.371; 6 -1.427,-0.8; 7 -1.427,-1.23; 8 -1.024,-1.23; 9 -0.62,-1.23; 10 -0.217,-1.23; 11 0.187,-1.23; 12 0.591,-1.23; 13 0.994,-1.23; 14 1.398,-1.23; 15 1.398,-0.8; 16 1.398,-0.371; 17 1.398,0.058; 18 1.398,0.487; 19 1.398,0.916; 20 1.398,1.346; 21 0.994,1.346; 22 0.591,1.346; 23 0.187,1.346; 24 -0.217,1.346; 25 -0.62,1.346; 26 -1.024,1.346 | hole 2: 0,10; 0,-10
DCK6-L = smd 0.864 x 0.305: 1 -0.927,0.65; 2 -0.927,0; 3 -0.927,-0.65; 4 0.927,-0.65; 5 0.927,0; 6 0.927,0.65
UDFN-6-MAXIM = smd 0.8 x 0.35: 1 -0.915,0.65; 2 -0.915,0; 3 -0.915,-0.65; 4 0.915,-0.65; 5 0.915,0; 6 0.915,0.65
UDFN-6-EXPOSED = smd 0.48 x 0.36: 1 -0.925,0.65; 2 -0.925,0; 3 -0.925,-0.65; 4 0.925,-0.65; 5 0.925,0; 6 0.925,0.65 | smd 0.71 x 1.4: EP 0,0
SOT-23-6 = smd 0.55 x 1.2: 1 -0.95,-1.3; 2 0,-1.3; 3 0.95,-1.3; 4 0.95,1.3; 5 0,1.3; 6 -0.95,1.3
AQFN73 = smd 0.3 x 0.3: A8 -1.25,3.25; A10 -0.75,3.25; A12 -0.25,3.25; A14 0.25,3.25; A16 0.75,3.25; A18 1.25,3.25; A20 1.75,3.25; A22 2.25,3.25; A23 2.75,3.25; AA24 3.25,-2.25; AB2 -2.75,-2.5; AC5 -2,-2.75; AC9 -1,-2.75; AC11 -0.5,-2.75; AC13 0,-2.75; AC15 0.5,-2.75; AC17 1,-2.75; AC19 1.5,-2.75; AC21 2,-2.75; AC24 3.25,-2.75; AD2 -2.75,-3.25; AD4 -2.25,-3.25; AD6 -1.75,-3.25; AD8 -1.25,-3.25; AD10 -0.75,-3.25; AD12 -0.25,-3.25; AD14 0.25,-3.25; AD16 0.75,-3.25; AD18 1.25,-3.25; AD20 1.75,-3.25; AD22 2.25,-3.25; AD23 2.75,-3.25; B1 -3.25,2.75; B3 -2.5,2.75; B5 -2,2.75; B7 -1.5,2.75; B9 -1,2.75; B11 -0.5,2.75; B13 0,2.75; B15 0.5,2.75; B17 1,2.75; B19 1.5,2.75; B24 3.25,2.75; C1 -3.25,2.25; D2 -2.75,2; D23 2.75,2; E24 3.25,1.75; F2 -2.75,1.5; F23 2.75,1.5; G1 -3.25,1.25; H2 -2.75,1; H23 2.75,1; J1 -3.25,0.75; J24 3.25,0.75; K2 -2.75,0.5; L1 -3.25,0.25; L24 3.25,0.25; M2 -2.75,0; N1 -3.25,-0.25; N24 3.25,-0.25; P2 -2.75,-0.5; P23 2.75,-0.5; R1 -3.25,-0.75; R24 3.25,-0.75; T2 -2.75,-1; T23 2.75,-1; U1 -3.25,-1.25; U24 3.25,-1.25; V23 2.75,-1.5; W1 -3.25,-1.75; W24 3.25,-1.75; Y2 -2.75,-2; Y23 2.75,-2 | smd 4.85 x 4.85: GND 0,0
TXC-7V = smd 1.4 x 1.2: 1 -1.1,-0.85; 2 1.1,-0.85; 3 1.1,0.85; 4 -1.1,0.85
ABS05 = smd 0.5 x 1: A -0.55,0; B 0.55,0
2-SMD = smd 1.092 x 1.905: 1 -1.245,0; 2 1.245,0

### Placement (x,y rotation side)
A2  2.97,27.47 0 top
BT1  20.45,32.89 180 bottom
BT2  13.59,15.75 90 bottom
C1  5.37,20.89 270 top
C2  2.83,20.89 270 top
C3  3.3,13.84 180 top
C4  6.48,15.37 90 top
C5  15.49,21.21 180 top
C6  16.76,20.19 180 top
C7  11.94,6.48 180 top
C8  4.28,18.91 180 top
C9  5.08,22.86 180 top
C10  22.64,53.98 90 top
C11  20.32,46.61 180 top
C12  11.21,16.22 180 top
C13  6.39,26.89 90 top
C14  9.4,27.81 90 top
C15  14.64,18.89 0 top
C16  6.9,17.37 180 top
C17  9.14,40.89 180 top
C18  10.67,53.72 0 top
C19  7.49,40.89 0 top
C20  14.64,17.88 0 top
C21  11.21,17.49 180 top
C22  20.32,2.67 270 top
C23  12.19,7.75 180 top
C24  13.72,24.51 90 top
C25  20.32,47.5 180 top
C26  24.13,53.2 180 top
C27  19.18,42.55 180 top
C28  19.18,36.58 180 top
C29  13.97,36.58 90 top
C30  18.03,5.21 270 top
C31  12.45,5.21 270 top
D1  25.15,48.64 270 top
D2  16.13,58.29 0 top
J1  2.54,33.66 90 top
L1  4.1,21.4 0 top
L2  12.23,15.46 0 top
L3  25.4,39.24 270 top
L4  12.74,16.99 90 top
L5  24,45.43 180 top
Q1  18.8,2.54 270 top
Q2  14.61,31.24 0 top
Q3  22.61,2.41 0 top
Q4  14.86,33.27 90 top
Q5  19.81,44.93 0 top
Q6  20.07,34.16 90 top
R1  13.59,57.15 180 top
R2  13.59,58.93 180 top
R3  13.59,58.04 180 top
R4  19.68,54.36 0 top
R5  20.95,5.84 270 top
R6  25.15,54.86 270 top
R7  17.78,7.49 270 top
R8  18.92,7.49 270 top
R9  10.79,29.34 90 top
R10  19.18,39.37 0 top
R11  20.95,54.86 270 top
R12  19.68,55.24 0 top
R13  19.68,56.77 180 top
R14  21.84,54.86 270 top
R15  19.18,40.77 180 top
R16  20.19,4.32 90 top
R17  17.53,1.65 90 top
R18  13.46,33.91 90 top
R19  20.19,14.35 270 top
R20  20.19,12.19 90 top
S1  24.51,58.42 180 top
TP1  23.24,5.97 0 top
TP2  22.23,5.97 0 top
TP3  15.37,14.22 180 top
TP4  17.91,13.21 0 top
TP5  17.27,14.48 0 top
TP6  11.56,11.3 0 top
TP7  4.83,30.35 0 top
TP8  7.11,29.08 0 top
TP9  5.59,34.8 0 top
TP10  18.29,11.56 0 top
TP11  16.51,1.14 0 top
TP12  6.99,34.8 0 top
TP13  12.83,11.94 180 top
TP14  16.89,10.54 180 top
TP15  14.22,12.19 0 top
TP16  13.21,14.1 0 top
TP17  0.76,37.72 0 top
TP18  9.27,29.72 0 top
TP19  7.75,34.04 0 top
TP20  9.53,33.15 0 top
TP21  21.97,4.45 0 top
TP22  0.76,10.16 0 top
TP23  25.78,52.7 0 top
TP24  9.65,46.23 180 bottom
TP25  23.11,36.7 0 top
TP26  0.76,12.83 0 top
TP27  0.76,11.43 0 top
TP28  9.65,47.24 0 bottom
TP29  9.65,48.26 0 bottom
U1  14.73,9.27 180 top
U2  20.45,51.15 90 top
U3  5.5,5.56 0 top
U4  8.89,47.24 0 top
U6  6.99,31.62 270 top
U7  22.23,39.37 90 top
U8  25.53,2.03 90 top
U9  11.43,32.77 180 top
U10  9.55,22.16 180 top
U$2  [UCB_CAL_200MIL]  18.03,24 0 top
X1  3.98,15.84 180 top
X3  14.99,20.19 180 top
X4  15.24,5.71 180 top

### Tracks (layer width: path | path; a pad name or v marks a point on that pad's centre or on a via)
!CAM_EN  (via drill 0.2)
  Top 0.102: Q2.2 v13.65,31.24 | v15.62,31.24 Q2.5
  Top 0.152: R18.1 13.46,32.51 13.72,32.26 v14.48,32.26 14.86,32.64 Q4.2 | v10.41,26.04 10.3,25.92 U10.AD10
  Bottom 0.152: 14.35,31.24 v15.62,31.24 | v14.48,32.26 14.35,32.13 14.35,31.24 | v10.41,26.04 10.41,28.07 12.45,30.1 13.34,30.1 13.72,30.48 13.72,31.18 v13.65,31.24 14.35,31.24
!FVLD
  Top 0.102: U6.1 7.63,33.39 6.48,34.54 6.48,34.8 | U4.5 6.86,46.86 6.48,46.48 6.48,34.8 | TP12.P$1 6.48,34.8
!LT_EN  (via drill 0.15, 0.2)
  Top 0.152: Q3.5 23.58,2.41 v23.62,2.46 | Q3.2 v21.59,2.41 21.59,2.92 20.83,3.68 20.19,3.68 | 18.8,3.68 19.43,3.68 | 19.43,3.68 20.19,3.68 | 19.43,3.68 19.43,8.26 18.67,9.02 18.67,10.14 18.29,10.52 | 18.29,10.52 TP10.P$1 | R16.1 20.19,3.68 | v17.83,10.97 18.29,10.52
  Top 0.203: 18.8,3.68 Q1.2
  Bottom 0.152: v23.62,2.46 23.62,2.41 v21.59,2.41 | U10.B11 10.05,19.19 9.78,18.92 9.78,13.72 12.95,10.54 17.4,10.54 v17.83,10.97
  other vias: 10.05,19.41
!LT_INT  (via drill 0.15, 0.2)
  Top 0.152: U8.4 26.18,3.29 25.53,3.94 23.29,3.94 22.38,4.85 | 22.38,4.85 R5.1 20.37,6.86 v20.32,6.86 | TP21.P$1 22.38,4.85
  Bottom 0.152: v20.32,6.86 17.14,6.86 15.62,8.38 13.46,8.38 9.53,12.32 9.53,19.38 U10.B13
  other vias: 9.55,19.41
!LVLD
  Top 0.102: U6.3 6.1,32.79 6.1,34.8 | U4.4 6.79,47.3 6.1,46.61 6.1,34.8 | TP9.P$1 6.1,34.8
!PIR_EN  (via drill 0.15, 0.2)
  Top 0.152: U10.B19 | U10.B19
  Top 0.203: Q1.5 v18.8,1.27 18.74,1.22 R17.1 16.59,1.22 TP11.P$1
  Bottom 0.152: U10.B19 8.13,19.33 8.13,6.29 13.15,1.27 v18.8,1.27
  other vias: 8.05,19.41
!RST  (via drill 0.15, 0.2)
  Top 0.152: U1.1 17.18,8.52 R7.1 17.2,7.93 v17.02,7.75 | J1.3 v4.06,33.66 4.57,34.16 4.57,36.58 3.43,37.72 TP17.P$1
  Route2 0.152: v17.02,7.75 17.4,8.13 17.4,13.59 11.68,19.3 11.68,23.88 11.43,24.13 9.78,24.13 9.55,24.36 U10.AC13
  Route15 0.152: v4.06,33.66 8.89,28.83 8.89,25.57 U10.AC13
  other vias: 9.55,24.91
!RTC_EXTR  (via drill 0.2)
  Top 0.152: U1.3 v17.01,9.52 v17.02,9.53 | S1.2 25.15,56.09 R6.1 25.73,55.3 v25.78,55.24
  Bottom 0.152: v17.02,9.53 18.16,9.53 20.57,11.94 20.57,25.27 26.54,31.24 26.54,54.48 v25.78,55.24
!RTC_IRQ1
  Top 0.152: U1.11 13.36,9.04 12.81,9.04 12.19,9.66 12.19,12 | U10.A16 8.64,18.74 8.64,15.56 12.19,12 | 12.19,12 12.26,11.94 TP13.P$1
!RTC_IRQ2
  Top 0.152: U10.A14 9.3,18.67 9.53,18.45 9.53,15.49 11.56,13.46 14.3,13.46 16.13,11.63 U1.4 16.37,10.02 TP14.P$1
!RTC_IRQ3  (via drill 0.15, 0.2)
  Top 0.152: v9.02,18.41 9.02,15.59 12.03,12.57 13.36,12.57 13.98,11.95 | U1.8 13.98,11.95 | 13.98,11.95 TP15.P$1
  Bottom 0.152: U10.B15 9.02,19.37 v9.02,18.41
  other vias: 9.05,19.41
!VBAT_PRI_ON  (via drill 0.2)
  Top 0.203: Q6.2 v20.07,33.15 | Q6.5 v20.07,35.18
  Top 0.254: v18.92,52.96 19.38,52.96 U2.10 | v20.07,35.18 18.67,35.18 17.02,36.83 v17.02,48.01
  Bottom 0.203: v20.07,35.18 v20.07,33.15
  Bottom 0.254: v17.02,48.01 17.02,51.05 v18.92,52.96
!VBAT_SEC_ON  (via drill 0.2)
  Top 0.152: Q5.2 18.83,44.93 v18.8,44.96 | Q5.5 20.7,44.93 v20.83,44.8
  Top 0.254: v19.3,53.72 19.68,53.72 19.95,53.46 U2.9 | v18.54,48.64 17.78,47.88 v17.78,44.58
  Bottom 0.254: v19.3,53.72 19.43,53.59 19.43,52.58 18.54,51.69 v18.54,48.64 | v17.78,44.58 18.16,44.96 v18.8,44.96
  Bottom 0.61: v20.83,44.8 20.67,44.96 v18.8,44.96
CAM_D0
  Top 0.102: U10.AD12 9.93,25.53 9.93,33.15 | 9.93,33.15 9.93,34.69 12.19,36.96 12.19,45.4 U4.17 | TP20.P$1 9.93,33.15
CAM_D1  (via drill 0.2)
  Top 0.102: U4.18 9.16,46.61 v9.02,46.61
  Bottom 0.102: v9.02,46.61 9.27,46.61 TP24.P$1
CAM_D2  (via drill 0.2)
  Top 0.102: U4.19 9.37,47.24 v8.89,47.24
  Bottom 0.102: v8.89,47.24 TP28.P$1
CAM_D3  (via drill 0.2)
  Top 0.102: U4.20 9.58,47.88 v9.02,47.88
  Bottom 0.102: v9.02,47.88 9.4,48.26 TP29.P$1
CAM_EN  (via drill 0.15, 0.2)
  Top 0.152: U9.6 12.38,30.8 v11.94,30.35 11.36,29.77 R9.2
  Bottom 0.152: U10.AC11 10.05,25.51 9.91,25.65 9.91,28.32 v11.94,30.35
  other vias: 10.05,24.91
CAM_INT  (via drill 0.15, 0.2)
  Top 0.152: U4.1 7.46,49.12 v7.49,49.15
  Bottom 0.152: U10.AC21 7.55,25.6 6.48,26.67 6.48,48.77 6.86,49.15 v7.49,49.15
  other vias: 7.55,24.91
CAM_SCL  (via drill 0.2)
  Top 0.152: Q2.3 14.02,30.73 v13.34,30.73 | U4.3 6.5,47.73 6.35,47.88 6.35,48.64 7.24,49.53 10.16,49.53 12.83,46.86 12.83,36.07 v13.08,35.81
  Bottom 0.152: v13.34,30.73 13.08,30.99 v13.08,35.81
CAM_SDA  (via drill 0.2)
  Top 0.152: v6.86,48.26 7.36,48.26 U4.2 | v8.51,49.91 10.79,49.91 14.86,45.85 14.86,35.71 15.62,34.95 15.62,32.18 Q2.6
  Bottom 0.152: v6.86,48.26 7.37,48.26 8,48.9 8,49.4 v8.51,49.91
CAM_TRIG  (via drill 0.15, 0.2)
  Top 0.152: U4.6 6.99,45.97 v6.86,45.97
  Bottom 0.152: v6.86,45.97 6.86,32.89 6.73,32.77 6.73,26.8 8.05,25.48 U10.AC19
  other vias: 8.05,24.91
FVLD
  Top 0.102: U6.6 7.8,30.53 7.8,29.08 | 7.8,29.08 U10.AD20 | TP8.P$1 7.8,29.08
GND  (via drill 0.2, 0.25, 0.41)
  Top 0.102: U10.F23 6.58,20.66 6.46,20.78 5.69,20.78 C1.2
  Top 0.152: U10.AD2 12.69,25.02 v12.83,25.02 | 7.62,20.65 7.73,20.76 v8.15,20.76 | 8.04,20.65 U10.GND 8.05,20.66 7.49,20.66 | v12.57,10.16 12.57,9.89 12.94,9.52 U1.10
  Top 0.203: U10.GND 11.05,20.66 U10.B7 11.18,19.28 11.18,18.29 10.78,17.89 C21.2 | U10.F23 7.49,20.66 | 7.62,20.65 8.04,20.65 v8.15,20.76 | U4.7 7.46,45.82 v7.24,45.59
  Top 0.254: U4.9 8.27,45.1 | 8.27,45.1 v8.13,44.96 | U4.10 8.67,45.5 8.27,45.1 | U4.11 9.08,45.15 v8.64,44.7
  Top 0.305: v2.54,19.68 2.83,19.97 C2.2
  Top 0.406: C4.1 5.13,14.93 X1.4
  other vias: 19.18,48.64 23.88,40.26 23.88,38.48 19.68,51.94 20.45,51.94 21.21,51.94 21.21,51.18 20.45,51.18 19.68,51.18 19.68,50.42 20.45,50.42 21.21,50.42 23.24,49.5 8.15,22.16 9.55,22.16 11,22.16 9.55,20.76 9.55,23.56 11,23.56 8.15,23.56 11,20.76 1.78,16.64 14.73,9.27 15.11,8.89 14.35,8.89 14.35,9.65 15.11,9.65 20.7,43.69 5.33,19.68 4.57,19.68 3.56,19.68 1.78,19.68 3.3,23.11 4.45,22.23 5.21,22.23 5.33,24.51 5.33,25.78 5.33,27.05 5.33,28.32 2.54,23.11 1.02,23.11 1.78,20.57 1.4,21.34 1.02,22.23 2.54,22.23 3.56,22.23 0.76,19.68 0.76,20.95 5.71,28.83 5.71,27.69 10.29,1.52 2.67,1.52 16.64,18.92 16.76,21.08 22.1,52.83 23.62,54.86 4.57,13.84 5.84,13.84 6.48,16.51 10.03,7.62 17.27,4.06 9.91,12.95 17.78,12.19 19.3,37.56 24.51,35.53 4.07,34.97 5.33,23.5 4.06,23.11 8.51,49.15 5.33,25.15 5.33,29.21 4.57,29.46 3.81,29.46 2.29,29.46 1.27,29.46 0.51,29.46 25.78,0.51 8.13,46.74 20.57,1.52 10.79,16.89 8,41.53 8.76,41.53 8.51,33.02 5.97,28.32 5.71,29.59 7.24,33.27 19.81,22.23 14.1,25.78 13.21,44.58 13.21,42.42 13.21,40.01 9.4,31.37 11.05,44.58 11.05,42.42 11.05,40.01 11.81,44.58 11.81,42.42 11.81,40.01 9.4,34.04 8.51,29.97 8.51,26.42 9.4,28.96 20.32,10.79 20.32,8.76 20.19,16.51 20.19,19.3 10.92,27.05 11.3,35.05
  pour Top (rank 2): 0,60 27,60 27,0 0,0
  pour Bottom (rank 2): 0,60 27,60 27,0 0,0
  pour Top (rank 2, no thermals): 4.11,26.71 4.11,28.23 5.4,28.23 5.4,26.7
  pour Route2 (rank 2): 0,60 0,0 27,0 27,60
LBST  (via drill 0.2)
  Top 0.152: L5.P$1 22.23,45.36 v22.23,43.69 | U10.U1 14.89,23.41 v14.98,23.5
  Top 0.203: 21.59,49.27 U2.20
  Top 0.406: L5.P$1 22.15,48.7 21.59,49.27
  Route2 0.152: v14.98,23.5 15.12,23.5 v18.67,27.05
  Bottom 0.152: v18.67,27.05 21.59,29.97 21.59,43.05 v22.23,43.69
LED_BLUE  (via drill 0.2)
  Top 0.152: U10.J1 13.79,21.41 v13.84,21.46 | v16.51,27.3 16.51,34.8 15.37,35.94 15.37,53.21 12.7,55.88 12.7,57.78 12.95,58.04 R3.2
  Bottom 0.152: v13.84,21.46 16.51,24.13 v16.51,27.3
LED_GREEN  (via drill 0.15, 0.2)
  Top 0.152: v16.13,26.92 16.13,34.8 15.11,35.81 15.11,53.09 12.45,55.75 12.45,58.29 13.08,58.93 R2.2
  Bottom 0.152: U10.K2 13.27,21.66 13.53,21.91 13.93,21.91 16.13,24.11 v16.13,26.92
  other vias: 12.3,21.66
LED_RED  (via drill 0.15, 0.2)
  Top 0.152: v16.89,26.92 16.89,34.8 15.62,36.07 15.62,53.34 13.21,55.75 13.21,57.1 R1.2
  Bottom 0.152: v16.89,26.92 16.89,23.88 13.97,20.95 12.5,20.95 U10.H2
  other vias: 12.3,21.16
LVLD
  Top 0.102: U10.AD22 7.3,28.01 6.33,28.97 6.33,30.35 | 6.33,30.35 U6.4 | TP7.P$1 6.33,30.35
MCLK
  Top 0.102: U10.AD18 8.13,25.58 8.13,34.04 | 8.13,34.04 8.13,34.42 10.67,36.96 10.67,46.06 U4.15 | TP19.P$1 8.13,34.04
MISO  (via drill 0.2)
  Top 0.152: U1.6 v14.98,11.43 v14.99,11.43 | TP4.P$1 18.07,13.21 | 18.07,13.21 18.41,13.55 18.41,21.21 16.89,22.73 13.13,22.73 U10.N1 | v16.34,12.49 17.36,12.49 18.07,13.21
  Bottom 0.152: v14.99,11.43 16.05,12.49 v16.34,12.49
MOSI  (via drill 0.2)
  Top 0.152: U1.9 13.38,11.1 v13.46,11.18 | 17.59,14.16 17.91,14.48 17.91,20.7 16.7,21.91 U10.L1 | TP5.P$1 17.59,14.16 | v16,13.72 17.14,13.72 17.59,14.16
  Bottom 0.152: v16,13.72 v13.46,11.18
N$1
  Top 0.203: U10.N24 5.97,22.41 C9.1
N$2
  Top 0.152: C15.1 13.2,19.91 U10.C1
N$3  (via drill 0.15, 0.2)
  Top 0.254: L2.1 11.65,15.61 C12.1 C21.1 11.68,17.52 v11.68,18.67 11.68,19.28 U10.B5
  Bottom 0.406: U10.E24 6.77,19.94 11.18,19.94 11.68,19.43 v11.68,18.67
  other vias: 6.3,20.41
N$4
  Top 0.152: 4.73,18.91 C8.1
  Top 0.203: U10.D23 6.45,19.8 6.13,19.8 5.24,18.91 4.73,18.91
N$5
  Top 0.102: U10.H23 6.56,21.16 6.45,21.05 5.64,21.05 C1.1
  Top 0.305: C1.1 4.61,21.32 arc-90 L1.2
N$6
  Top 0.305: L1.1 arc-90 3.59,21.32 C2.1 arc-90 1.64,22.51 A2.S1
N$7
  cutout Route2: 5.14,23.4 5.14,29.12 0.06,29.12 0.06,23.4
N$8
  Top 0.203: C3.2 X1.3 2.15,14.99 1.32,15.82 1.32,16.83 2.04,17.55 4.44,17.55 U10.B24
N$9
  Top 0.203: U10.A23 5.1,17.2 5.08,17.2 X1.1 5.58,16.69 C4.2
N$10  (via drill 0.2)
  Top 0.254: U4.23 9.08,49.08 v9.14,49.15 | v9.65,53.72 C18.1 | U4.13 10.03,45.87 | 10.03,45.87 v10.03,45.47 | U4.14 10.14,45.87 10.03,45.87
  Bottom 0.254: v9.65,53.72 9.14,53.21 v9.14,49.15 10.03,49.15 10.67,48.51 10.67,45.97 10.16,45.47 v10.03,45.47
N$11
  cutout Top: 6.86,21.84 6.86,20.07 2.29,20.07 2.29,21.84
N$12
  Top 0.203: R10.2 22.48,39.37 22.88,39.77 U7.4
N$13  (via drill 0.2)
  Top 0.203: U6.5 6.99,29.97 v7.11,29.84 | C19.1 6.99,40.97
  Top 0.254: U4.12 9.53,45.97 9.53,40.95 | Q4.6 14.22,33.98 14.22,34.92 v14.1,35.05
  Top 0.305: 6.99,40.97 6.99,44.58 7.87,45.46 U4.8 | U9.1 12.38,34.99 v12.32,35.05 | 9.53,40.95 C17.1
  Top 0.813: C19.1 7.06,39.8 7.24,39.62 v8.38,39.62 9.02,39.62 9.58,40.18 C17.1
  Route15 0.406: v12.32,35.05 v14.1,35.05
  Bottom 0.152: 10.79,38.99 10.73,39.05
  Bottom 0.203: v7.11,29.84 7.11,32.57 7.64,33.11 7.64,33.43 10.79,36.58
  Bottom 0.813: 10.73,39.05 10.16,39.62 v8.38,39.62 | 10.79,38.99 10.79,36.58 v12.32,35.05
N$14
  Top 0.203: U7.6 21.09,40.77 R15.1
N$15
  Top 0.152: D2.2 15.85,57.15 R1.1
N$17
  Top 0.152: R2.1 14.22,58.73 D2.4
N$18
  Top 0.254: R14.2 21.82,54.43 | 21.82,54.43 R11.1 | U2.7 20.95,53.56 21.82,54.43
N$19
  Top 0.152: D2.3 14.2,57.86 R3.1
N$20
  Top 0.203: U8.1 20.15,1.11 Q1.6
N$23
  Top 0.203: Q1.3 18.24,2.96 18.16,3.05
  Top 0.406: U3.VCC 3.68,7.34 3.68,5.59 8.26,1.02 14.86,1.02 16.89,3.05 18.16,3.05
N$25
  Top 0.203: U1.14 14.48,7.24 14.22,6.99 12.88,6.99 C7.1
N$26
  Top 0.203: U1.16 15.48,7.25 16.48,6.25 X4.1 17.96,5.71 C30.1
N$27
  Top 0.203: U1.15 14.98,7.24 14.99,7.24 14.22,6.48 13.97,6.48 13.99,6.45 X4.2 12.52,5.71 C31.1
N$32
  Top 0.254: U2.8 20.45,54.03 R4.2 20.88,54.36 R11.2
N$35
  cutout Route15: 5.14,23.4 5.14,29.12 0.06,29.12 0.06,23.4
N$38
  cutout Top: 0.06,23.4 0.06,29.12 2.84,29.12 5.14,29.12 5.14,28.23 4.11,28.23 4.11,26.71 5.14,26.7 5.14,23.4
N$39
  cutout Bottom: 5.14,23.4 5.14,29.12 0.06,29.12 0.06,23.4
N$44
  Top 0.254: L4.2 12.74,18.73 12.72,18.73 U10.B3
N$45
  Top 0.203: Q5.4 20.24,44.11 19.81,43.69 18.54,43.69 18.29,43.94 18.29,45.21 18.54,45.47 19.2,45.47 Q5.1
N$49
  Top 0.254: L4.1 12.74,15.54 L2.2
N$51
  Top 0.152: Q3.3 22.18,1.82 22.61,1.4 23.88,1.4 24.38,1.91 24.38,2.46 U8.6
N$52
  Top 0.152: Q3.6 23.82,3.56 25.15,3.56 25.53,3.17 U8.5
N$53
  Top 0.152: Q6.4 20.45,34.59
  Top 0.203: Q6.1 19.59,33.61 19.59,32.89 19.84,32.64 21.02,32.64 21.32,32.94 21.32,34.21 20.94,34.59 20.45,34.59
N$57
  Top 0.254: R13.2 R12.1 17.78,53.77 17.78,51.94 18.07,51.65 U2.12
N$58
  Top 0.254: U2.11 18.35,52.51 18.35,53.45 R4.1 20.12,55.22 R12.2
PCLKO
  Top 0.102: U10.AD16 8.89,25.5 8.89,29.06 8.89,29.72 | 8.89,29.72 8.89,34.42 11.43,36.96 11.43,45.73 U4.16 | TP18.P$1 8.89,29.72
PIR_OUT
  Top 0.152: U3.OUT 2.54,4.92 2.54,7.62 | U10.A20 7.87,18.83 7.87,12.95 2.54,7.62 | TP22.P$1 2.54,8.38 2.54,7.62
RTC_CS  (via drill 0.15, 0.2)
  Top 0.152: U1.12 12.81,8.52 11.56,9.78 TP6.P$1 11.56,12.15 8.72,14.99 v8.64,14.99
  Bottom 0.152: U10.B17 8.64,19.32 v8.64,14.99
  other vias: 8.55,19.41
SCK  (via drill 0.15, 0.2)
  Top 0.152: U1.7 v14.48,11.43 | TP3.P$1 15.37,13.59 v15.98,12.98 16.87,12.98 18.16,14.27 18.16,20.95 16.76,22.35 v13.34,22.35
  Bottom 0.152: v14.48,11.43 14.48,11.56 15.9,12.98 v15.98,12.98 | U10.M2 12.49,22.35 v13.34,22.35
  other vias: 12.3,22.16
SCL  (via drill 0.15, 0.2)
  Top 0.152: v11.94,26.29 15.62,26.29 | 15.62,26.29 16.36,26.29 20.95,21.7 20.95,11.81 | v21.08,4.06 22.18,2.96 Q3.1 | 20.95,11.81 20.95,8.13 19.94,7.11 19.94,6.1 v20.19,5.84 | v22.65,5.12 22.23,5.54 TP2.P$1 | R20.1 20.25,11.81 20.95,11.81 | Q2.4 15.62,30.3 15.62,26.29
  Bottom 0.152: v20.19,5.84 20.19,4.95 v21.08,4.06 22.14,5.12 v22.65,5.12 | U10.AC9 v11.94,26.29
  other vias: 10.55,24.91
SDA  (via drill 0.2)
  Top 0.152: v19.81,5.46 19.68,5.59 19.68,14.73 | 19.68,14.73 19.68,21.59 15.88,25.4 12.77,25.4 12.63,25.54 12.26,25.91 11.3,25.91 | TP1.P$1 23.24,4.95 v23.88,4.32 | U10.AD8 10.8,25.66 11.05,25.91 11.3,25.91 | R19.1 20.14,14.73 19.68,14.73 | Q2.1 13.87,31.59 13.72,31.75 13.46,31.75 12.95,31.24 12.95,30.23 11.3,28.57 11.3,25.91
  Top 0.203: Q3.4 23.24,1.85 v23.69,1.85
  Bottom 0.152: v19.81,5.46 19.81,3.56 21.97,1.4 23.24,1.4 v23.69,1.85 24,2.16 24,4.19 v23.88,4.32
SW  (via drill 0.2)
  Top 0.152: v16.76,23.11 16.64,22.99 12.88,22.99 U10.R1
  Bottom 0.152: v24,36.2 24,30.35 v16.76,23.11
  pour Top (isolate 0.203, no thermals): 22.1,38.86 22.1,35.94 26.92,35.94 26.92,37.59 22.35,37.59 22.35,38.86
SWDCLK  (via drill 0.15, 0.2)
  Top 0.152: J1.4 1.91,33.53 v1.4,33.02
  Route15 0.152: U10.AA24 6.37,24.41 6.73,24.77 6.73,29.7 3.79,32.64 1.78,32.64 v1.4,33.02
  other vias: 6.3,24.41
SWDIO  (via drill 0.15, 0.2)
  Top 0.152: v1.4,31.88 J1.2
  Route15 0.152: U10.AC24 6.35,24.96 6.35,29.72 3.94,32.13 1.65,32.13 v1.4,31.88
  other vias: 6.3,24.91
VBAT  (via drill 0.15, 0.2, 0.3)
  Top 0.152: U1.5 15.48,11.29 v15.62,11.43
  Top 0.203: Q6.6 19.63,34.67 19.43,34.67
  Top 0.254: U2.14 18.26,50.65 v17.53,49.91
  Top 0.305: v17.02,35.81 18.16,34.67 19.43,34.67
  Top 0.813: v17.53,49.91 16.26,48.64 16.26,36.58 v17.02,35.81
  Route15 0.152: v15.62,11.43 14.86,12.19
  Route15 0.203: U10.A10 11.17,18.03 12.19,18.03
  Route15 1.016: BT2.2 14.35,28.45 16.51,30.61 16.51,35.31 v17.02,35.81
  other vias: 10.3,18.91
  pour Route15 (no thermals): 12.06,30.1 15.11,30.1 15.11,1.14 12.06,1.14
VBAT_OK  (via drill 0.15, 0.2)
  Top 0.152: v17.91,51.18 17.94,51.15 U2.13
  Bottom 0.152: v17.91,51.18 17.91,48.01 15.24,45.34 15.24,32.64 16.13,31.75 16.13,30.86 15.75,30.48 15.75,25.53 13.38,23.16 U10.T2
  other vias: 12.3,23.16
VCC  (via drill 0.2, 0.3, 0.41)
  Top 0.152: D2.1 16.13,58.29 v14.99,58.29 | TP26.P$1 v0.76,13.59 | v25.78,54.48 25.73,54.43 R6.2 | J1.1 3.56,32 v3.56,31.5 | R20.2 v20.19,13.21 R19.2 | Q4.1 14.05,32.85 v13.97,32.77 | U10.W1
  Top 0.203: C13.1 6.38,25.72 6.66,25.44 6.76,25.44 U10.AD23 | 7.31,17.38 C16.1 | R7.2 17.81,7.05 R8.2 | U1.13 13.86,7.75 12.7,7.75 C23.1 | Q1.1 19.2,3.02 v19.65,3.02 20.24,3.02 C22.1 | Q1.4 17.56,2.12 R17.2 17.45,2.16 v16.89,2.16 | R5.2 21.08,5.28 v21.08,4.7 20.25,4.7 R16.2
  Top 0.254: 13.24,18.98 13.23,18.98 U10.B1 | U10.A22 7.3,18.29 | 7.31,17.38 7.3,17.39 7.3,18.29 | v6.86,18.29 7.3,18.29 | 12.7,7.75 12.07,7.12 v11.43,7.12 | R8.2 18.8,6.93 v18.8,6.22 | U10.AD14 v9.3,26.7 9.3,27.28 C14.1 | C13.1 5.79,26.46 v5.74,26.41
  Top 0.305: 13.24,18.98 13.24,18.73 13.5,18.48 | R18.2 13.46,35.42 C29.1 14.73,35.16 v14.73,34.8 | v10.54,30.48 10.48,30.54 U9.4 U9.5
  Top 0.406: 14.1,17.88 C20.1 | 14.1,17.88 13.5,18.48 | U10.Y2 12.55,24.16 U10.W1 12.97,24.08 C24.1 14.99,24.08 15.42,24.51 v15.49,24.51 | v16.13,17.02 14.96,17.02 14.72,17.26 14.71,17.26 14.1,17.88
  other vias: 20.19,37.72 21.08,36.45 20.83,37.21
  pour Top (isolate 0.203, no thermals): 20.7,38.73 21.59,38.73 21.59,35.94 19.68,35.94 19.68,38.23 20.7,38.23
  pour Route15 (rank 2): 0,60 27,60 27,0 0,0
VOC_SAMP_VSTOR  (via drill 0.2)
  Top 0.203: v20.95,48.39 20.95,48.62 U2.19
  Top 0.254: U2.3 22.2,51.17 23.69,51.17 23.73,51.21 v23.84,51.21
  Top 0.406: v20.95,48.39 20.95,47.7 C25.1
  Bottom 0.406: v20.95,48.39 23.78,51.21 v23.84,51.21
  pour Top (no thermals): 20.57,48.13 21.21,48.13 21.21,45.21 20.07,45.21 20.07,45.72 20.57,46.23
VREF_SAMP
  Top 0.406: U2.4 22.93,51.65 22.93,53.25 C10.1
VSEC  (via drill 0.2)
  Top 0.152: U10.A8 10.8,18.67 10.29,18.16 10.29,15.75 11.3,14.73 15.11,14.73 v17.53,17.14 | v19.05,24.26 19.05,31.79 BT1.+
  Top 0.254: U2.18 20.45,48.39 v20.19,48.13
  Bottom 0.152: v17.53,17.14 17.53,17.17 19.05,18.69 v19.05,24.26
  Bottom 0.813: v20.19,48.13 15.88,43.81 15.88,34.97 BT1.+
VSOL  (via drill 0.15, 0.2)
  Top 0.406: U2.2 24.5,50.65
  Bottom 0.152: U10.B9 11.05,18.91 11.05,18.41 11.3,18.16 12.57,18.16 13.34,18.92 v15.88,18.92 17.14,20.19 17.14,22.99 25.15,30.99 D1.+
  other vias: 10.55,19.41
  pour Top (no thermals): 24.26,53.51 24.26,44.16 27.02,44.16 27.02,53.51
VSW  (via drill 0.2, 0.41)
  Top 0.152: v18.8,44.16 19.21,44.58 Q5.3
  Top 0.203: Q6.3 20.83,33.33 v20.83,33.15
  Top 0.406: R15.2 18.53,41.24 C27.1
  Bottom 0.61: v18.8,44.16 20.8,42.16
  Bottom 0.813: 20.8,42.16 v20.7,42.16 18.03,39.5 18.03,37.72 19.68,36.07 20.18,36.07 20.83,35.42 v20.83,33.15
  pour Top (isolate 0.203, no thermals): 22.1,39.88 22.1,41.4 19.81,41.4 19.81,42.8 26.92,42.8 26.92,40.89 22.35,40.89 22.35,39.88
WDI
  Top 0.152: U1.2 17.53,9.02 | 17.53,9.02 17.83,9.02 R8.1 | 17.53,9.02 17.53,10.74 14.55,13.72 13.21,13.72 | U10.A12 9.91,18.8 9.91,15.62 11.81,13.72 13.21,13.72 | TP16.P$1 13.21,13.72
XL1
  Top 0.102: U10.D2 12.56,20.16 12.66,20.25 13.34,20.25 14.1,19.49 14.83,19.49 X3.A
  Top 0.203: X3.A 15.61,20.12 15.69,20.19 C6.2
XL2
  Top 0.102: U10.F2 12.55,20.66 12.66,20.55 14.08,20.55 X3.B
  Top 0.203: C5.2 14.44,20.58 X3.B

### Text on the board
bPlace: SECONDARY
tNames: RESET | SOLAR | Permacam / Neal Jackson / 10/19 | VCC | GND | SOLAR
